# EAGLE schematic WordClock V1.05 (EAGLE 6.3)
PROJECT_LINE1: WordClock; PROJECT_REVISION: 1.05

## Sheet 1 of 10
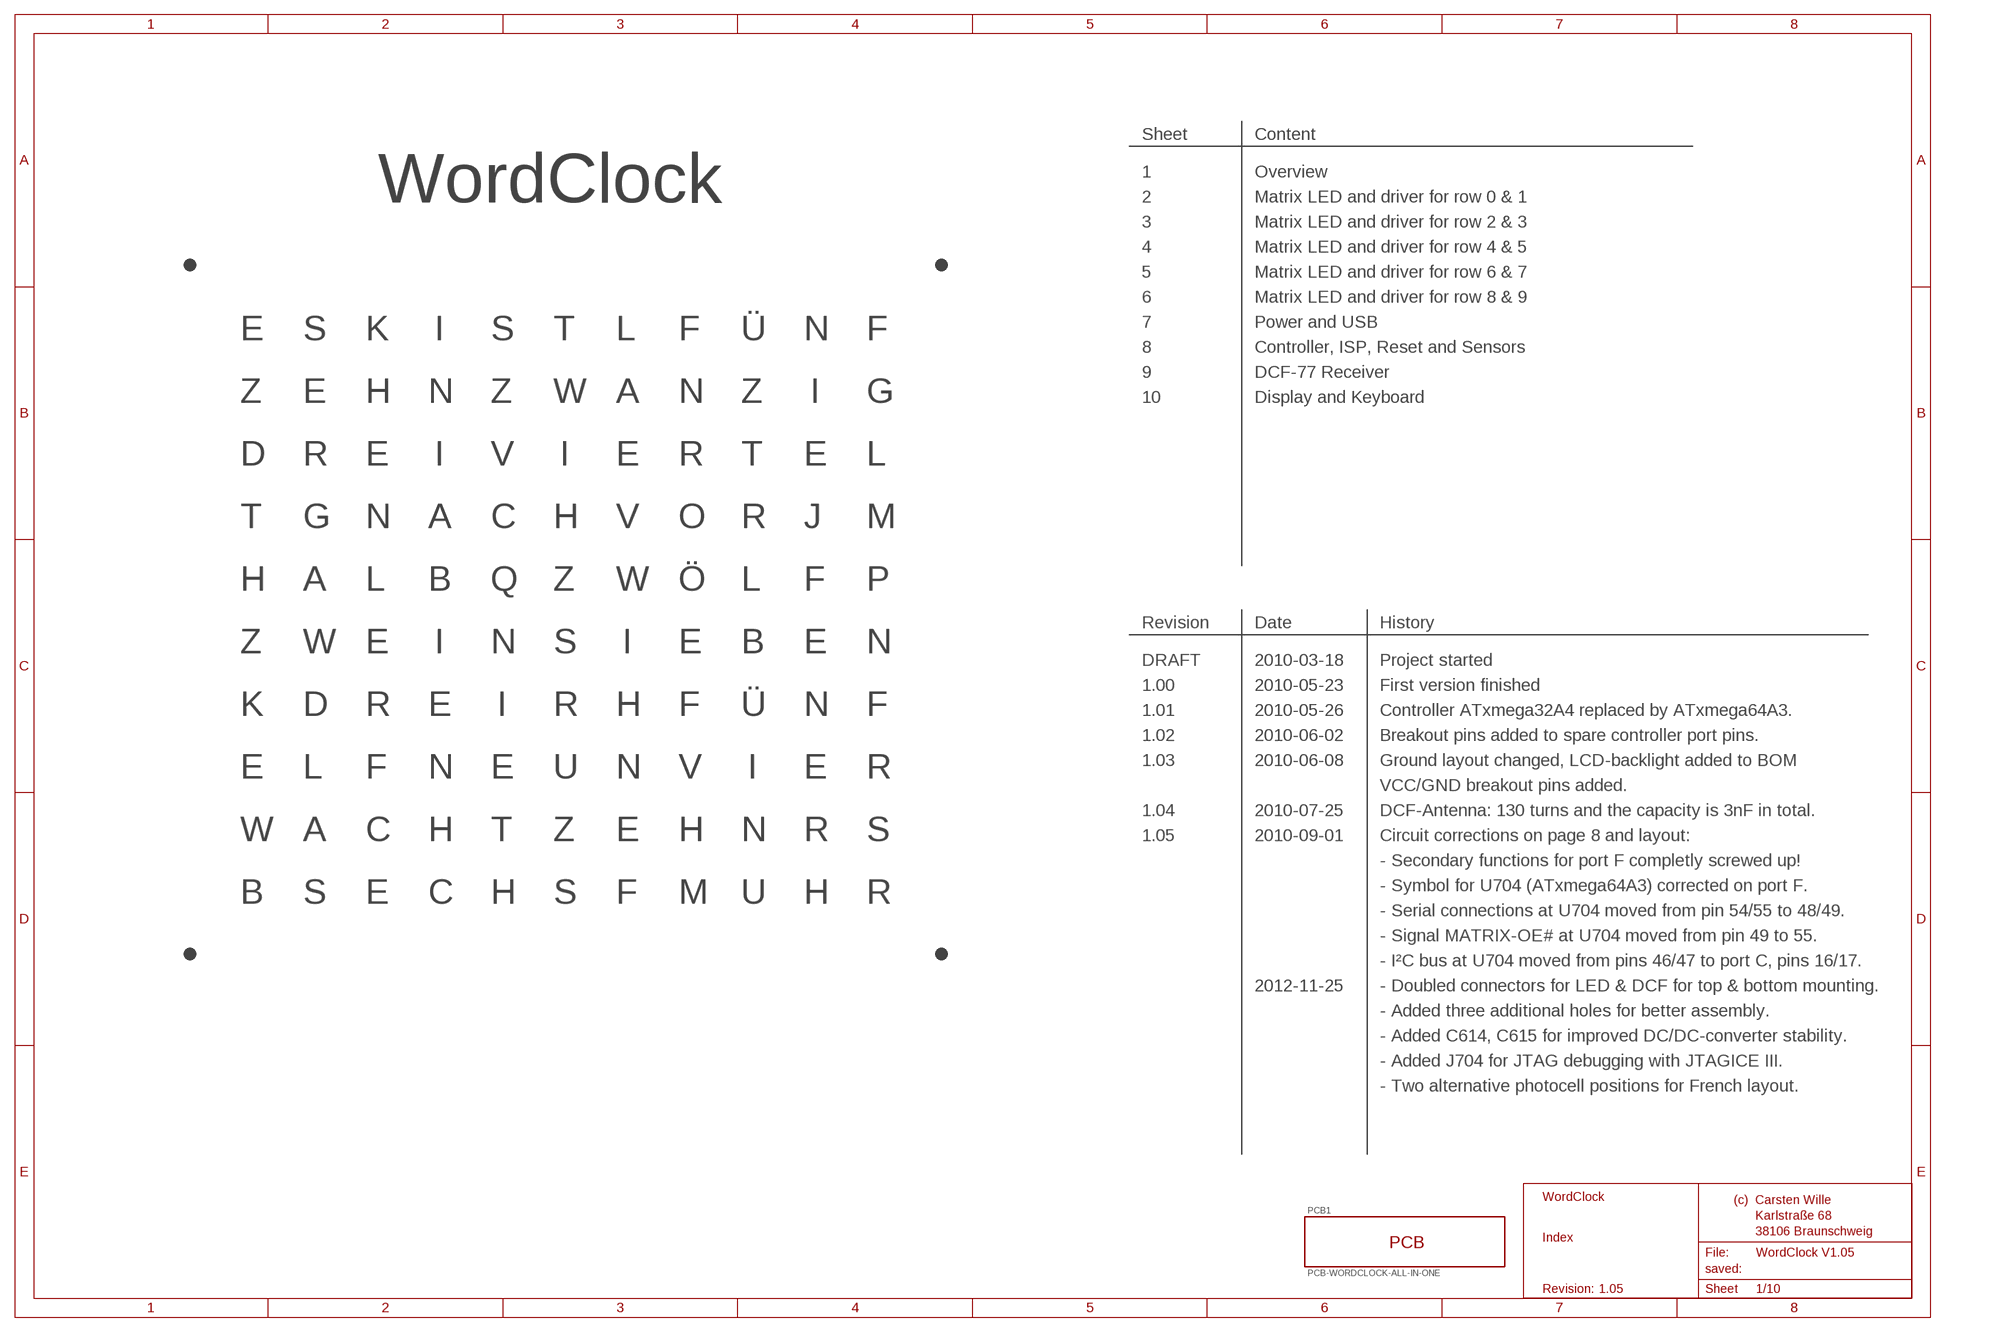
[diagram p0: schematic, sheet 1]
BLATT2 (BLATT-A3-LANDSCAPE_CW): SHEET_LINE1: Index

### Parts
PCB1  PCB-WORDCLOCK-ALL-IN-ONE  PCBWORDCLOCK-ALL-IN-ONE  [WORDCLOCK_S]

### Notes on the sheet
- Sheet | Content
- 1 | Overview
- WordClock | 2 | Matrix LED and driver for row 0 & 1
- 3 | Matrix LED and driver for row 2 & 3
- 4 | Matrix LED and driver for row 4 & 5
- 5 | Matrix LED and driver for row 6 & 7
- 6 | Matrix LED and driver for row 8 & 9
- 7 | Power and USB
- E | S | K | I | S | T | L | F | Ü | N | F
- 8 | Controller, ISP, Reset and Sensors
- 9 | DCF-77 Receiver
- Z | E | H | N | Z | W | A | N | Z | I | G | 10 | Display and Keyboard
- D | R | E | I | V | I | E | R | T | E | L
- T | G | N | A | C | H | V | O | R | J | M
- H | A | L | B | Q | Z | W | Ö | L | F | P
- Revision | Date | History
- Z | W | E | I | N | S | I | E | B | E | N
- DRAFT | 2010-03-18 | Project started
- 1.00 | 2010-05-23 | First version finished
- K | D | R | E | I | R | H | F | Ü | N | F | 1.01 | 2010-05-26 | Controller ATxmega32A4 replaced by ATxmega64A3.
- 1.02 | 2010-06-02 | Breakout pins added to spare controller port pins.
- 1.03 | 2010-06-08 | Ground layout changed, LCD-backlight added to BOM
- E | L | F | N | E | U | N | V | I | E | R
- VCC/GND breakout pins added.
- 1.04 | 2010-07-25 | DCF-Antenna: 130 turns and the capacity is 3nF in total.
- W | A | C | H | T | Z | E | H | N | R | S | 1.05 | 2010-09-01 | Circuit corrections on page 8 and layout:
- - Secondary functions for port F completly screwed up!
- - Symbol for U704 (ATxmega64A3) corrected on port F.
- B | S | E | C | H | S | F | M | U | H | R
- - Serial connections at U704 moved from pin 54/55 to 48/49.
- - Signal MATRIX-OE# at U704 moved from pin 49 to 55.
- - I²C bus at U704 moved from pins 46/47 to port C, pins 16/17.
- 2012-11-25 | - Doubled connectors for LED & DCF for top & bottom mounting.
- - Added three additional holes for better assembly.
- - Added C614, C615 for improved DC/DC-converter stability.
- - Added J704 for JTAG debugging with JTAGICE III.
- - Two alternative photocell positions for French layout.

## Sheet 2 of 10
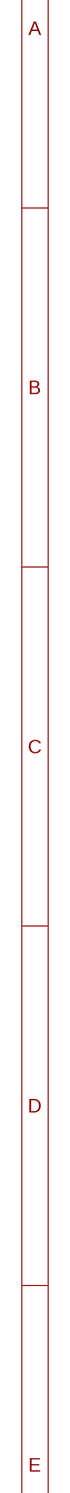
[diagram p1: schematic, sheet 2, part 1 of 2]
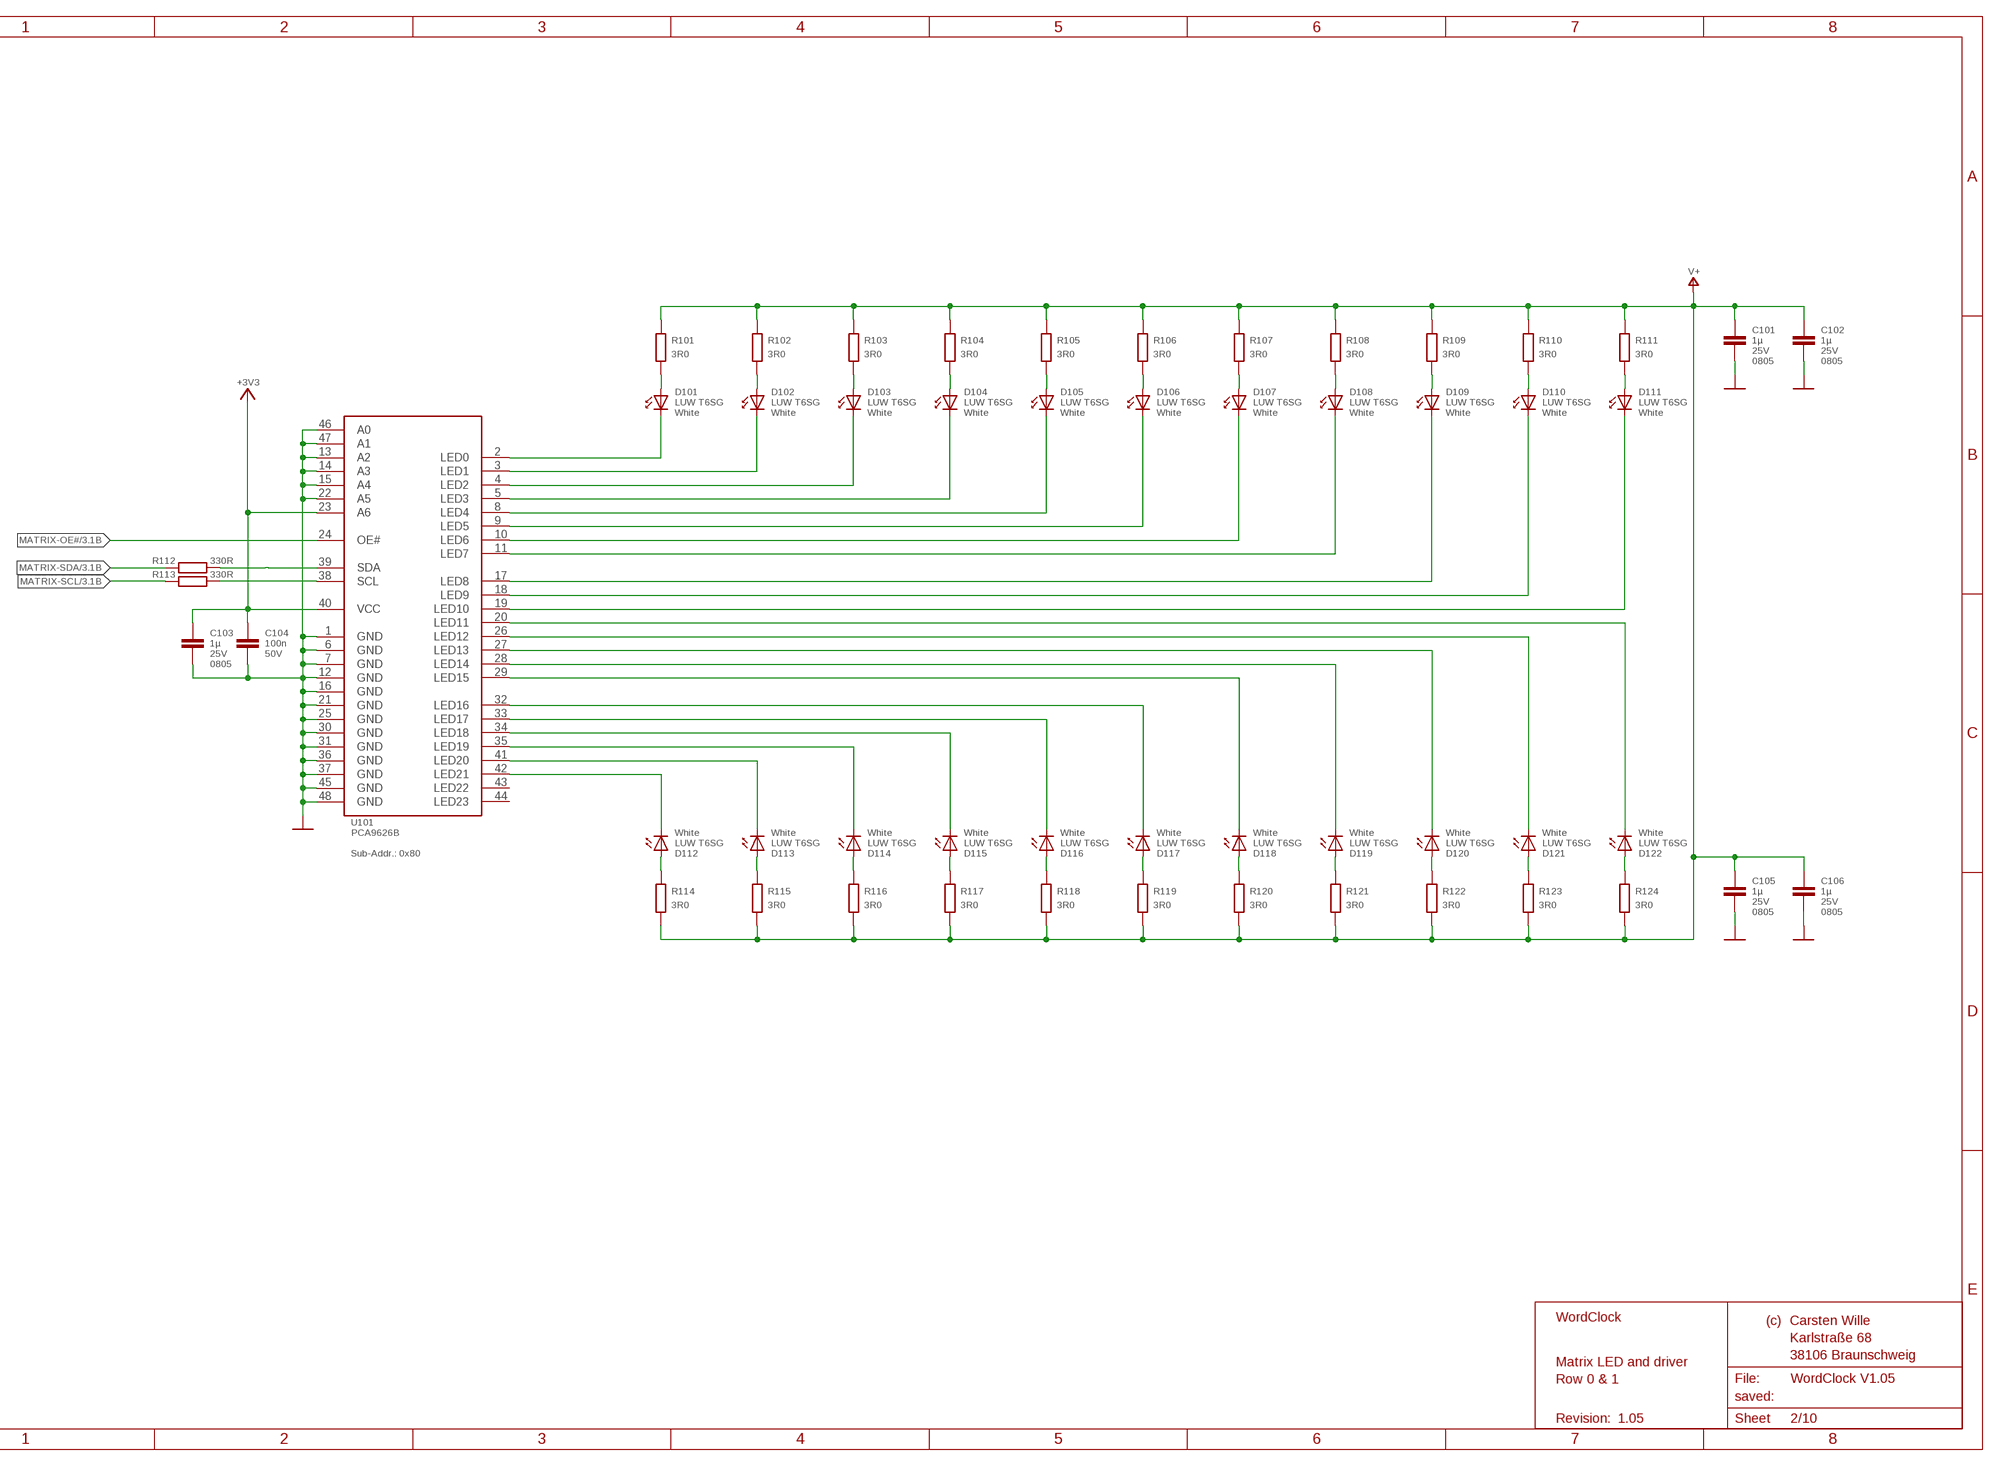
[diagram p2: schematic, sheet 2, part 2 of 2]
BLATT1 (BLATT-A3-LANDSCAPE_CW): SHEET_LINE1: Matrix LED and driver; SHEET_LINE2: Row 0 & 1

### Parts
C101  1E-6-1U-0805  [C0805]
C102  1E-6-1U-0805  [C0805]
C103  1E-6-1U-0805  [C0805]
C104  1E-9-100N-0603  [C0603]
C105  1E-6-1U-0805  [C0805]
C106  1E-6-1U-0805  [C0805]
D101  TOPLED-LUW  [P-LCC-2]
D102  TOPLED-LUW  [P-LCC-2]
D103  TOPLED-LUW  [P-LCC-2]
D104  TOPLED-LUW  [P-LCC-2]
D105  TOPLED-LUW  [P-LCC-2]
D106  TOPLED-LUW  [P-LCC-2]
D107  TOPLED-LUW  [P-LCC-2]
D108  TOPLED-LUW  [P-LCC-2]
D109  TOPLED-LUW  [P-LCC-2]
D110  TOPLED-LUW  [P-LCC-2]
D111  TOPLED-LUW  [P-LCC-2]
D112  TOPLED-LUW  [P-LCC-2]
D113  TOPLED-LUW  [P-LCC-2]
D114  TOPLED-LUW  [P-LCC-2]
D115  TOPLED-LUW  [P-LCC-2]
D116  TOPLED-LUW  [P-LCC-2]
D117  TOPLED-LUW  [P-LCC-2]
D118  TOPLED-LUW  [P-LCC-2]
D119  TOPLED-LUW  [P-LCC-2]
D120  TOPLED-LUW  [P-LCC-2]
D121  TOPLED-LUW  [P-LCC-2]
D122  TOPLED-LUW  [P-LCC-2]
R101  1E0-3,0R-0603  [R0603]
R102  1E0-3,0R-0603  [R0603]
R103  1E0-3,0R-0603  [R0603]
R104  1E0-3,0R-0603  [R0603]
R105  1E0-3,0R-0603  [R0603]
R106  1E0-3,0R-0603  [R0603]
R107  1E0-3,0R-0603  [R0603]
R108  1E0-3,0R-0603  [R0603]
R109  1E0-3,0R-0603  [R0603]
R110  1E0-3,0R-0603  [R0603]
R111  1E0-3,0R-0603  [R0603]
R112  1E2-330R-0603  [R0603]
R113  1E2-330R-0603  [R0603]
R114  1E0-3,0R-0603  [R0603]
R115  1E0-3,0R-0603  [R0603]
R116  1E0-3,0R-0603  [R0603]
R117  1E0-3,0R-0603  [R0603]
R118  1E0-3,0R-0603  [R0603]
R119  1E0-3,0R-0603  [R0603]
R120  1E0-3,0R-0603  [R0603]
R121  1E0-3,0R-0603  [R0603]
R122  1E0-3,0R-0603  [R0603]
R123  1E0-3,0R-0603  [R0603]
R124  1E0-3,0R-0603  [R0603]
U101  PCA9626  [LQFP48]

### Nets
+3V3: C103.1 C104.1 U101.23(A6) U101.40(VCC) ; also sheet 3,4,5,6,7,8
GND: C101.2 C102.2 C103.2 C104.2 C105.2 C106.2 U101.1(GND) U101.6(GND) U101.7(GND) U101.12(GND) U101.13(A2) U101.14(A3) U101.15(A4) U101.16(GND) U101.21(GND) U101.22(A5) U101.25(GND) U101.30(GND) U101.31(GND) U101.36(GND) U101.37(GND) U101.45(GND) U101.46(A0) U101.47(A1) U101.48(GND) ; also sheet 3,4,5,6,7,8
LED0@U1: D101.C U101.2(LED0)
LED1@U1: D102.C U101.3(LED1)
LED2@U1: D103.C U101.4(LED2)
LED3@U1: D104.C U101.5(LED3)
LED4@U1: D105.C U101.8(LED4)
LED5@U1: D106.C U101.9(LED5)
LED6@U1: D107.C U101.10(LED6)
LED7@U1: D108.C U101.11(LED7)
LED8@U1: D109.C U101.17(LED8)
LED9@U1: D110.C U101.18(LED9)
LED10@U1: D111.C U101.19(LED10)
LED11@U1: D122.C U101.20(LED11)
LED12@U1: D121.C U101.26(LED12)
LED13@U1: D120.C U101.27(LED13)
LED14@U1: D119.C U101.28(LED14)
LED15@U1: D118.C U101.29(LED15)
LED16@U1: D117.C U101.32(LED16)
LED17@U1: D116.C U101.33(LED17)
LED18@U1: D115.C U101.34(LED18)
LED19@U1: D114.C U101.35(LED19)
LED20@U1: D113.C U101.41(LED20)
LED21@U1: D112.C U101.42(LED21)
MATRIX-OE#: U101.24(OE#) ; also sheet 3,4,5,6,8
MATRIX-SCL: R113.1 ; also sheet 3,4,5,6,8
MATRIX-SDA: R112.1 ; also sheet 3,4,5,6,8
R1@U1: D101.A R101.2
R2@U1: D102.A R102.2
R3@U1: D103.A R103.2
R4@U1: D104.A R104.2
R5@U1: D105.A R105.2
R6@U1: D106.A R106.2
R7@U1: D107.A R107.2
R8@U1: D108.A R108.2
R9@U1: D109.A R109.2
R10@U1: D110.A R110.2
R11@U1: D111.A R111.2
R12@U1: D112.A R114.1
R13@U1: D113.A R115.1
R14@U1: D114.A R116.1
R15@U1: D115.A R117.1
R16@U1: D116.A R118.1
R17@U1: D117.A R119.1
R18@U1: D118.A R120.1
R19@U1: D119.A R121.1
R20@U1: D120.A R122.1
R21@U1: D121.A R123.1
R22@U1: D122.A R124.1
SCL@U1: R113.2 U101.38(SCL)
SDA@U1: R112.2 U101.39(SDA)
V+: C101.1 C102.1 C105.1 C106.1 R101.1 R102.1 R103.1 R104.1 R105.1 R106.1 R107.1 R108.1 R109.1 R110.1 R111.1 R114.2 R115.2 R116.2 R117.2 R118.2 R119.2 R120.2 R121.2 R122.2 R123.2 R124.2 ; also sheet 3,4,5,6,7
Unconnected: U101.43(LED22) U101.44(LED23)

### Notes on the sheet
- Sub-Addr.: 0x80

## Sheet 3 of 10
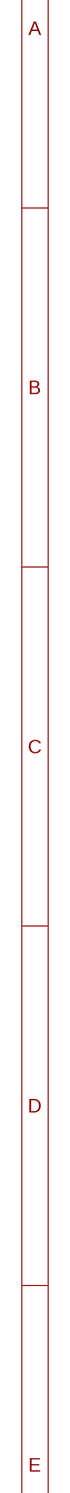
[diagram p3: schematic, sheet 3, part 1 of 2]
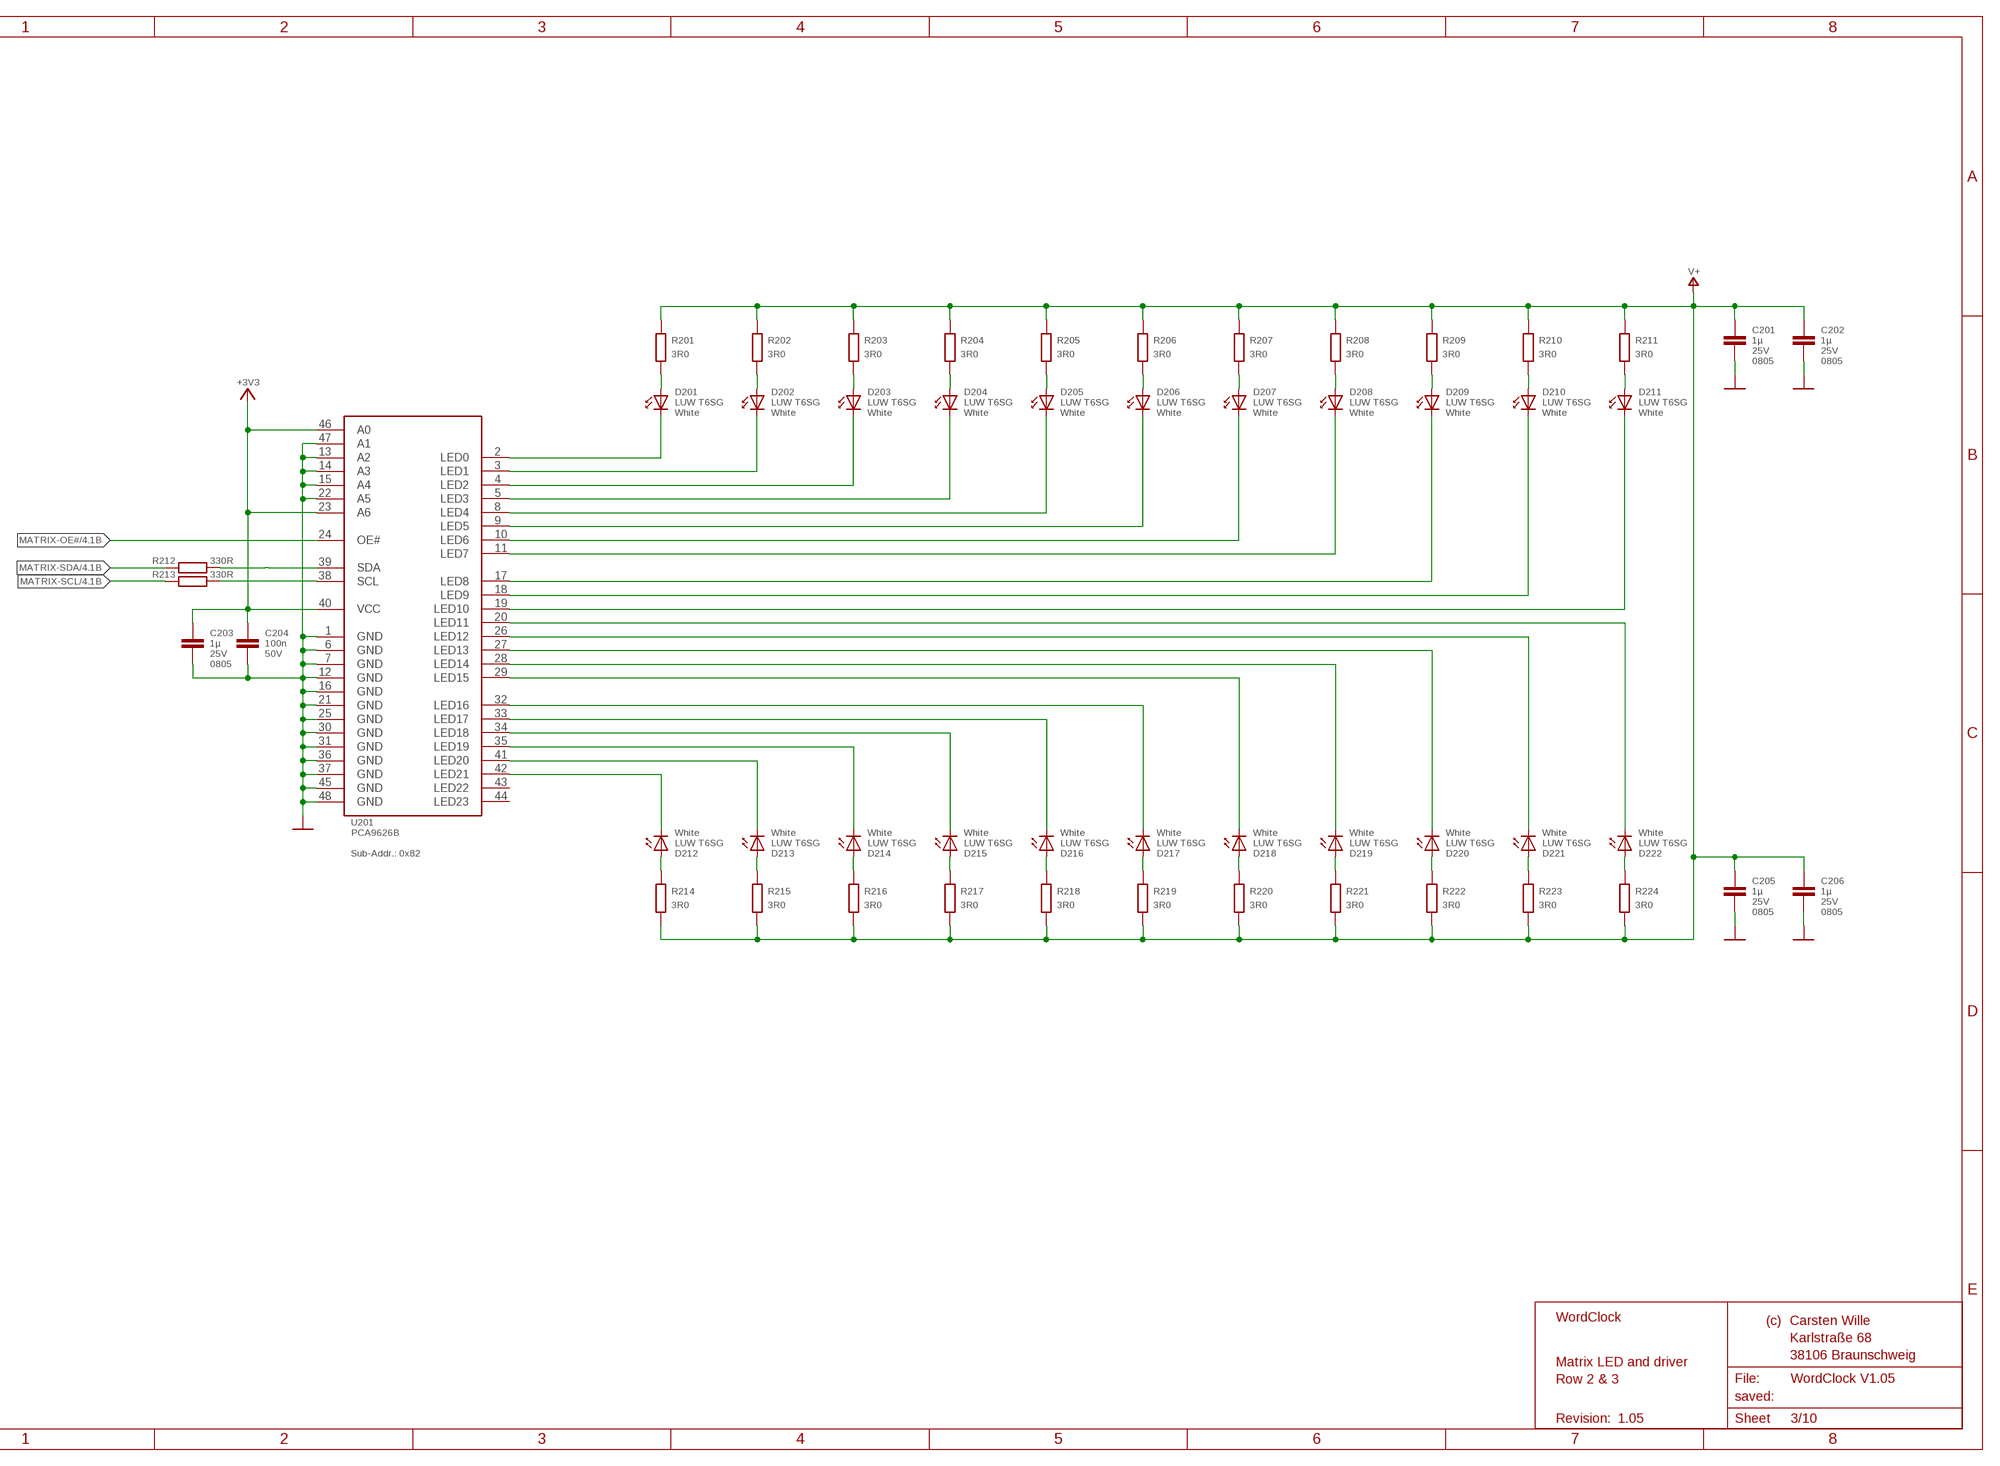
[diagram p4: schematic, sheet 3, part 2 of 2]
BLATT3 (BLATT-A3-LANDSCAPE_CW): SHEET_LINE1: Matrix LED and driver; SHEET_LINE2: Row 2 & 3

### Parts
C201  1E-6-1U-0805  [C0805]
C202  1E-6-1U-0805  [C0805]
C203  1E-6-1U-0805  [C0805]
C204  1E-9-100N-0603  [C0603]
C205  1E-6-1U-0805  [C0805]
C206  1E-6-1U-0805  [C0805]
D201  TOPLED-LUW  [P-LCC-2]
D202  TOPLED-LUW  [P-LCC-2]
D203  TOPLED-LUW  [P-LCC-2]
D204  TOPLED-LUW  [P-LCC-2]
D205  TOPLED-LUW  [P-LCC-2]
D206  TOPLED-LUW  [P-LCC-2]
D207  TOPLED-LUW  [P-LCC-2]
D208  TOPLED-LUW  [P-LCC-2]
D209  TOPLED-LUW  [P-LCC-2]
D210  TOPLED-LUW  [P-LCC-2]
D211  TOPLED-LUW  [P-LCC-2]
D212  TOPLED-LUW  [P-LCC-2]
D213  TOPLED-LUW  [P-LCC-2]
D214  TOPLED-LUW  [P-LCC-2]
D215  TOPLED-LUW  [P-LCC-2]
D216  TOPLED-LUW  [P-LCC-2]
D217  TOPLED-LUW  [P-LCC-2]
D218  TOPLED-LUW  [P-LCC-2]
D219  TOPLED-LUW  [P-LCC-2]
D220  TOPLED-LUW  [P-LCC-2]
D221  TOPLED-LUW  [P-LCC-2]
D222  TOPLED-LUW  [P-LCC-2]
R201  1E0-3,0R-0603  [R0603]
R202  1E0-3,0R-0603  [R0603]
R203  1E0-3,0R-0603  [R0603]
R204  1E0-3,0R-0603  [R0603]
R205  1E0-3,0R-0603  [R0603]
R206  1E0-3,0R-0603  [R0603]
R207  1E0-3,0R-0603  [R0603]
R208  1E0-3,0R-0603  [R0603]
R209  1E0-3,0R-0603  [R0603]
R210  1E0-3,0R-0603  [R0603]
R211  1E0-3,0R-0603  [R0603]
R212  1E2-330R-0603  [R0603]
R213  1E2-330R-0603  [R0603]
R214  1E0-3,0R-0603  [R0603]
R215  1E0-3,0R-0603  [R0603]
R216  1E0-3,0R-0603  [R0603]
R217  1E0-3,0R-0603  [R0603]
R218  1E0-3,0R-0603  [R0603]
R219  1E0-3,0R-0603  [R0603]
R220  1E0-3,0R-0603  [R0603]
R221  1E0-3,0R-0603  [R0603]
R222  1E0-3,0R-0603  [R0603]
R223  1E0-3,0R-0603  [R0603]
R224  1E0-3,0R-0603  [R0603]
U201  PCA9626  [LQFP48]

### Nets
+3V3: C203.1 C204.1 U201.23(A6) U201.40(VCC) U201.46(A0) ; also sheet 2,4,5,6,7,8
GND: C201.2 C202.2 C203.2 C204.2 C205.2 C206.2 U201.1(GND) U201.6(GND) U201.7(GND) U201.12(GND) U201.13(A2) U201.14(A3) U201.15(A4) U201.16(GND) U201.21(GND) U201.22(A5) U201.25(GND) U201.30(GND) U201.31(GND) U201.36(GND) U201.37(GND) U201.45(GND) U201.47(A1) U201.48(GND) ; also sheet 2,4,5,6,7,8
LED0@U2: D201.C U201.2(LED0)
LED1@U2: D202.C U201.3(LED1)
LED2@U2: D203.C U201.4(LED2)
LED3@U2: D204.C U201.5(LED3)
LED4@U2: D205.C U201.8(LED4)
LED5@U2: D206.C U201.9(LED5)
LED6@U2: D207.C U201.10(LED6)
LED7@U2: D208.C U201.11(LED7)
LED8@U2: D209.C U201.17(LED8)
LED9@U2: D210.C U201.18(LED9)
LED10@U2: D211.C U201.19(LED10)
LED11@U2: D222.C U201.20(LED11)
LED12@U2: D221.C U201.26(LED12)
LED13@U2: D220.C U201.27(LED13)
LED14@U2: D219.C U201.28(LED14)
LED15@U2: D218.C U201.29(LED15)
LED16@U2: D217.C U201.32(LED16)
LED17@U2: D216.C U201.33(LED17)
LED18@U2: D215.C U201.34(LED18)
LED19@U2: D214.C U201.35(LED19)
LED20@U2: D213.C U201.41(LED20)
LED21@U2: D212.C U201.42(LED21)
MATRIX-OE#: U201.24(OE#) ; also sheet 2,4,5,6,8
MATRIX-SCL: R213.1 ; also sheet 2,4,5,6,8
MATRIX-SDA: R212.1 ; also sheet 2,4,5,6,8
R1@U2: D201.A R201.2
R2@U2: D202.A R202.2
R3@U2: D203.A R203.2
R4@U2: D204.A R204.2
R5@U2: D205.A R205.2
R6@U2: D206.A R206.2
R7@U2: D207.A R207.2
R8@U2: D208.A R208.2
R9@U2: D209.A R209.2
R10@U2: D210.A R210.2
R11@U2: D211.A R211.2
R12@U2: D212.A R214.1
R13@U2: D213.A R215.1
R14@U2: D214.A R216.1
R15@U2: D215.A R217.1
R16@U2: D216.A R218.1
R17@U2: D217.A R219.1
R18@U2: D218.A R220.1
R19@U2: D219.A R221.1
R20@U2: D220.A R222.1
R21@U2: D221.A R223.1
R22@U2: D222.A R224.1
SCL@U2: R213.2 U201.38(SCL)
SDA@U2: R212.2 U201.39(SDA)
V+: C201.1 C202.1 C205.1 C206.1 R201.1 R202.1 R203.1 R204.1 R205.1 R206.1 R207.1 R208.1 R209.1 R210.1 R211.1 R214.2 R215.2 R216.2 R217.2 R218.2 R219.2 R220.2 R221.2 R222.2 R223.2 R224.2 ; also sheet 2,4,5,6,7
Unconnected: U201.43(LED22) U201.44(LED23)

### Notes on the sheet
- Sub-Addr.: 0x82

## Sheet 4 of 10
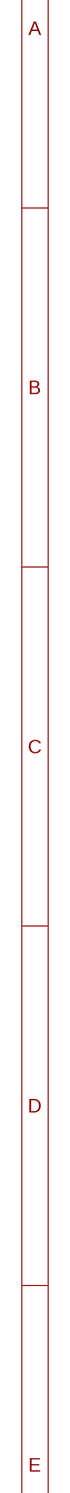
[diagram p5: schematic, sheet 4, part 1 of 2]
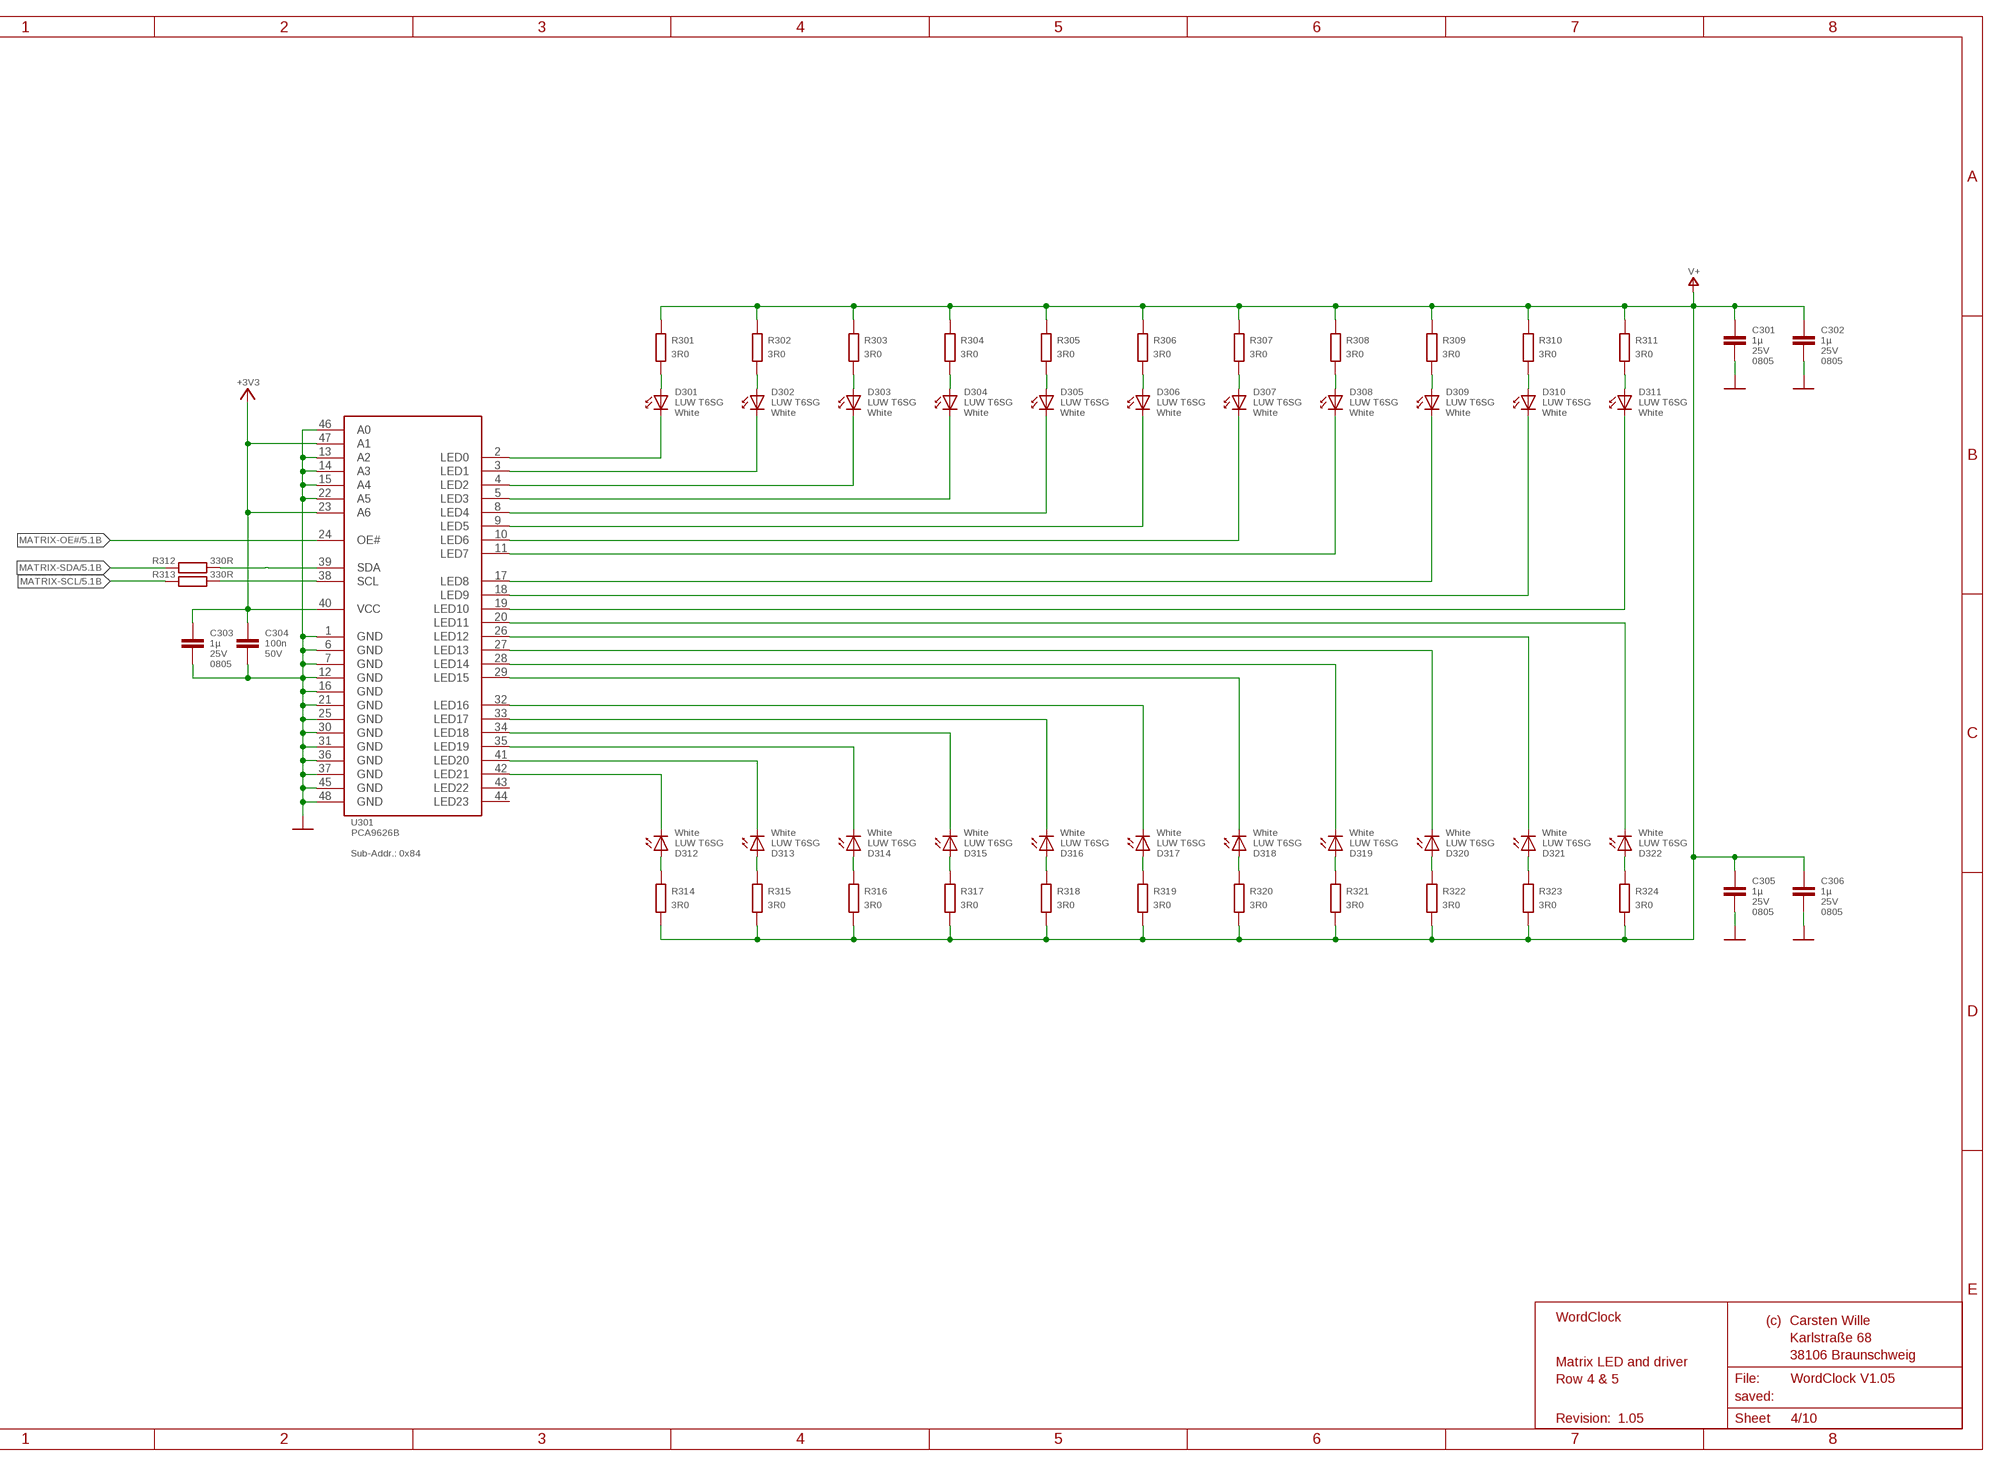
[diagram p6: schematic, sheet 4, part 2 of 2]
BLATT4 (BLATT-A3-LANDSCAPE_CW): SHEET_LINE1: Matrix LED and driver; SHEET_LINE2: Row 4 & 5

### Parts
C301  1E-6-1U-0805  [C0805]
C302  1E-6-1U-0805  [C0805]
C303  1E-6-1U-0805  [C0805]
C304  1E-9-100N-0603  [C0603]
C305  1E-6-1U-0805  [C0805]
C306  1E-6-1U-0805  [C0805]
D301  TOPLED-LUW  [P-LCC-2]
D302  TOPLED-LUW  [P-LCC-2]
D303  TOPLED-LUW  [P-LCC-2]
D304  TOPLED-LUW  [P-LCC-2]
D305  TOPLED-LUW  [P-LCC-2]
D306  TOPLED-LUW  [P-LCC-2]
D307  TOPLED-LUW  [P-LCC-2]
D308  TOPLED-LUW  [P-LCC-2]
D309  TOPLED-LUW  [P-LCC-2]
D310  TOPLED-LUW  [P-LCC-2]
D311  TOPLED-LUW  [P-LCC-2]
D312  TOPLED-LUW  [P-LCC-2]
D313  TOPLED-LUW  [P-LCC-2]
D314  TOPLED-LUW  [P-LCC-2]
D315  TOPLED-LUW  [P-LCC-2]
D316  TOPLED-LUW  [P-LCC-2]
D317  TOPLED-LUW  [P-LCC-2]
D318  TOPLED-LUW  [P-LCC-2]
D319  TOPLED-LUW  [P-LCC-2]
D320  TOPLED-LUW  [P-LCC-2]
D321  TOPLED-LUW  [P-LCC-2]
D322  TOPLED-LUW  [P-LCC-2]
R301  1E0-3,0R-0603  [R0603]
R302  1E0-3,0R-0603  [R0603]
R303  1E0-3,0R-0603  [R0603]
R304  1E0-3,0R-0603  [R0603]
R305  1E0-3,0R-0603  [R0603]
R306  1E0-3,0R-0603  [R0603]
R307  1E0-3,0R-0603  [R0603]
R308  1E0-3,0R-0603  [R0603]
R309  1E0-3,0R-0603  [R0603]
R310  1E0-3,0R-0603  [R0603]
R311  1E0-3,0R-0603  [R0603]
R312  1E2-330R-0603  [R0603]
R313  1E2-330R-0603  [R0603]
R314  1E0-3,0R-0603  [R0603]
R315  1E0-3,0R-0603  [R0603]
R316  1E0-3,0R-0603  [R0603]
R317  1E0-3,0R-0603  [R0603]
R318  1E0-3,0R-0603  [R0603]
R319  1E0-3,0R-0603  [R0603]
R320  1E0-3,0R-0603  [R0603]
R321  1E0-3,0R-0603  [R0603]
R322  1E0-3,0R-0603  [R0603]
R323  1E0-3,0R-0603  [R0603]
R324  1E0-3,0R-0603  [R0603]
U301  PCA9626  [LQFP48]

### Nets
+3V3: C303.1 C304.1 U301.23(A6) U301.40(VCC) U301.47(A1) ; also sheet 2,3,5,6,7,8
GND: C301.2 C302.2 C303.2 C304.2 C305.2 C306.2 U301.1(GND) U301.6(GND) U301.7(GND) U301.12(GND) U301.13(A2) U301.14(A3) U301.15(A4) U301.16(GND) U301.21(GND) U301.22(A5) U301.25(GND) U301.30(GND) U301.31(GND) U301.36(GND) U301.37(GND) U301.45(GND) U301.46(A0) U301.48(GND) ; also sheet 2,3,5,6,7,8
LED0@U3: D301.C U301.2(LED0)
LED1@U3: D302.C U301.3(LED1)
LED2@U3: D303.C U301.4(LED2)
LED3@U3: D304.C U301.5(LED3)
LED4@U3: D305.C U301.8(LED4)
LED5@U3: D306.C U301.9(LED5)
LED6@U3: D307.C U301.10(LED6)
LED7@U3: D308.C U301.11(LED7)
LED8@U3: D309.C U301.17(LED8)
LED9@U3: D310.C U301.18(LED9)
LED10@U3: D311.C U301.19(LED10)
LED11@U3: D322.C U301.20(LED11)
LED12@U3: D321.C U301.26(LED12)
LED13@U3: D320.C U301.27(LED13)
LED14@U3: D319.C U301.28(LED14)
LED15@U3: D318.C U301.29(LED15)
LED16@U3: D317.C U301.32(LED16)
LED17@U3: D316.C U301.33(LED17)
LED18@U3: D315.C U301.34(LED18)
LED19@U3: D314.C U301.35(LED19)
LED20@U3: D313.C U301.41(LED20)
LED21@U3: D312.C U301.42(LED21)
MATRIX-OE#: U301.24(OE#) ; also sheet 2,3,5,6,8
MATRIX-SCL: R313.1 ; also sheet 2,3,5,6,8
MATRIX-SDA: R312.1 ; also sheet 2,3,5,6,8
R1@U3: D301.A R301.2
R2@U3: D302.A R302.2
R3@U3: D303.A R303.2
R4@U3: D304.A R304.2
R5@U3: D305.A R305.2
R6@U3: D306.A R306.2
R7@U3: D307.A R307.2
R8@U3: D308.A R308.2
R9@U3: D309.A R309.2
R10@U3: D310.A R310.2
R11@U3: D311.A R311.2
R12@U3: D312.A R314.1
R13@U3: D313.A R315.1
R14@U3: D314.A R316.1
R15@U3: D315.A R317.1
R16@U3: D316.A R318.1
R17@U3: D317.A R319.1
R18@U3: D318.A R320.1
R19@U3: D319.A R321.1
R20@U3: D320.A R322.1
R21@U3: D321.A R323.1
R22@U3: D322.A R324.1
SCL@U3: R313.2 U301.38(SCL)
SDA@U3: R312.2 U301.39(SDA)
V+: C301.1 C302.1 C305.1 C306.1 R301.1 R302.1 R303.1 R304.1 R305.1 R306.1 R307.1 R308.1 R309.1 R310.1 R311.1 R314.2 R315.2 R316.2 R317.2 R318.2 R319.2 R320.2 R321.2 R322.2 R323.2 R324.2 ; also sheet 2,3,5,6,7
Unconnected: U301.43(LED22) U301.44(LED23)

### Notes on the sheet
- Sub-Addr.: 0x84

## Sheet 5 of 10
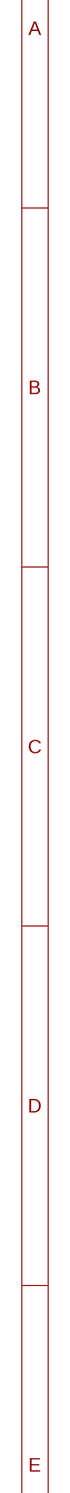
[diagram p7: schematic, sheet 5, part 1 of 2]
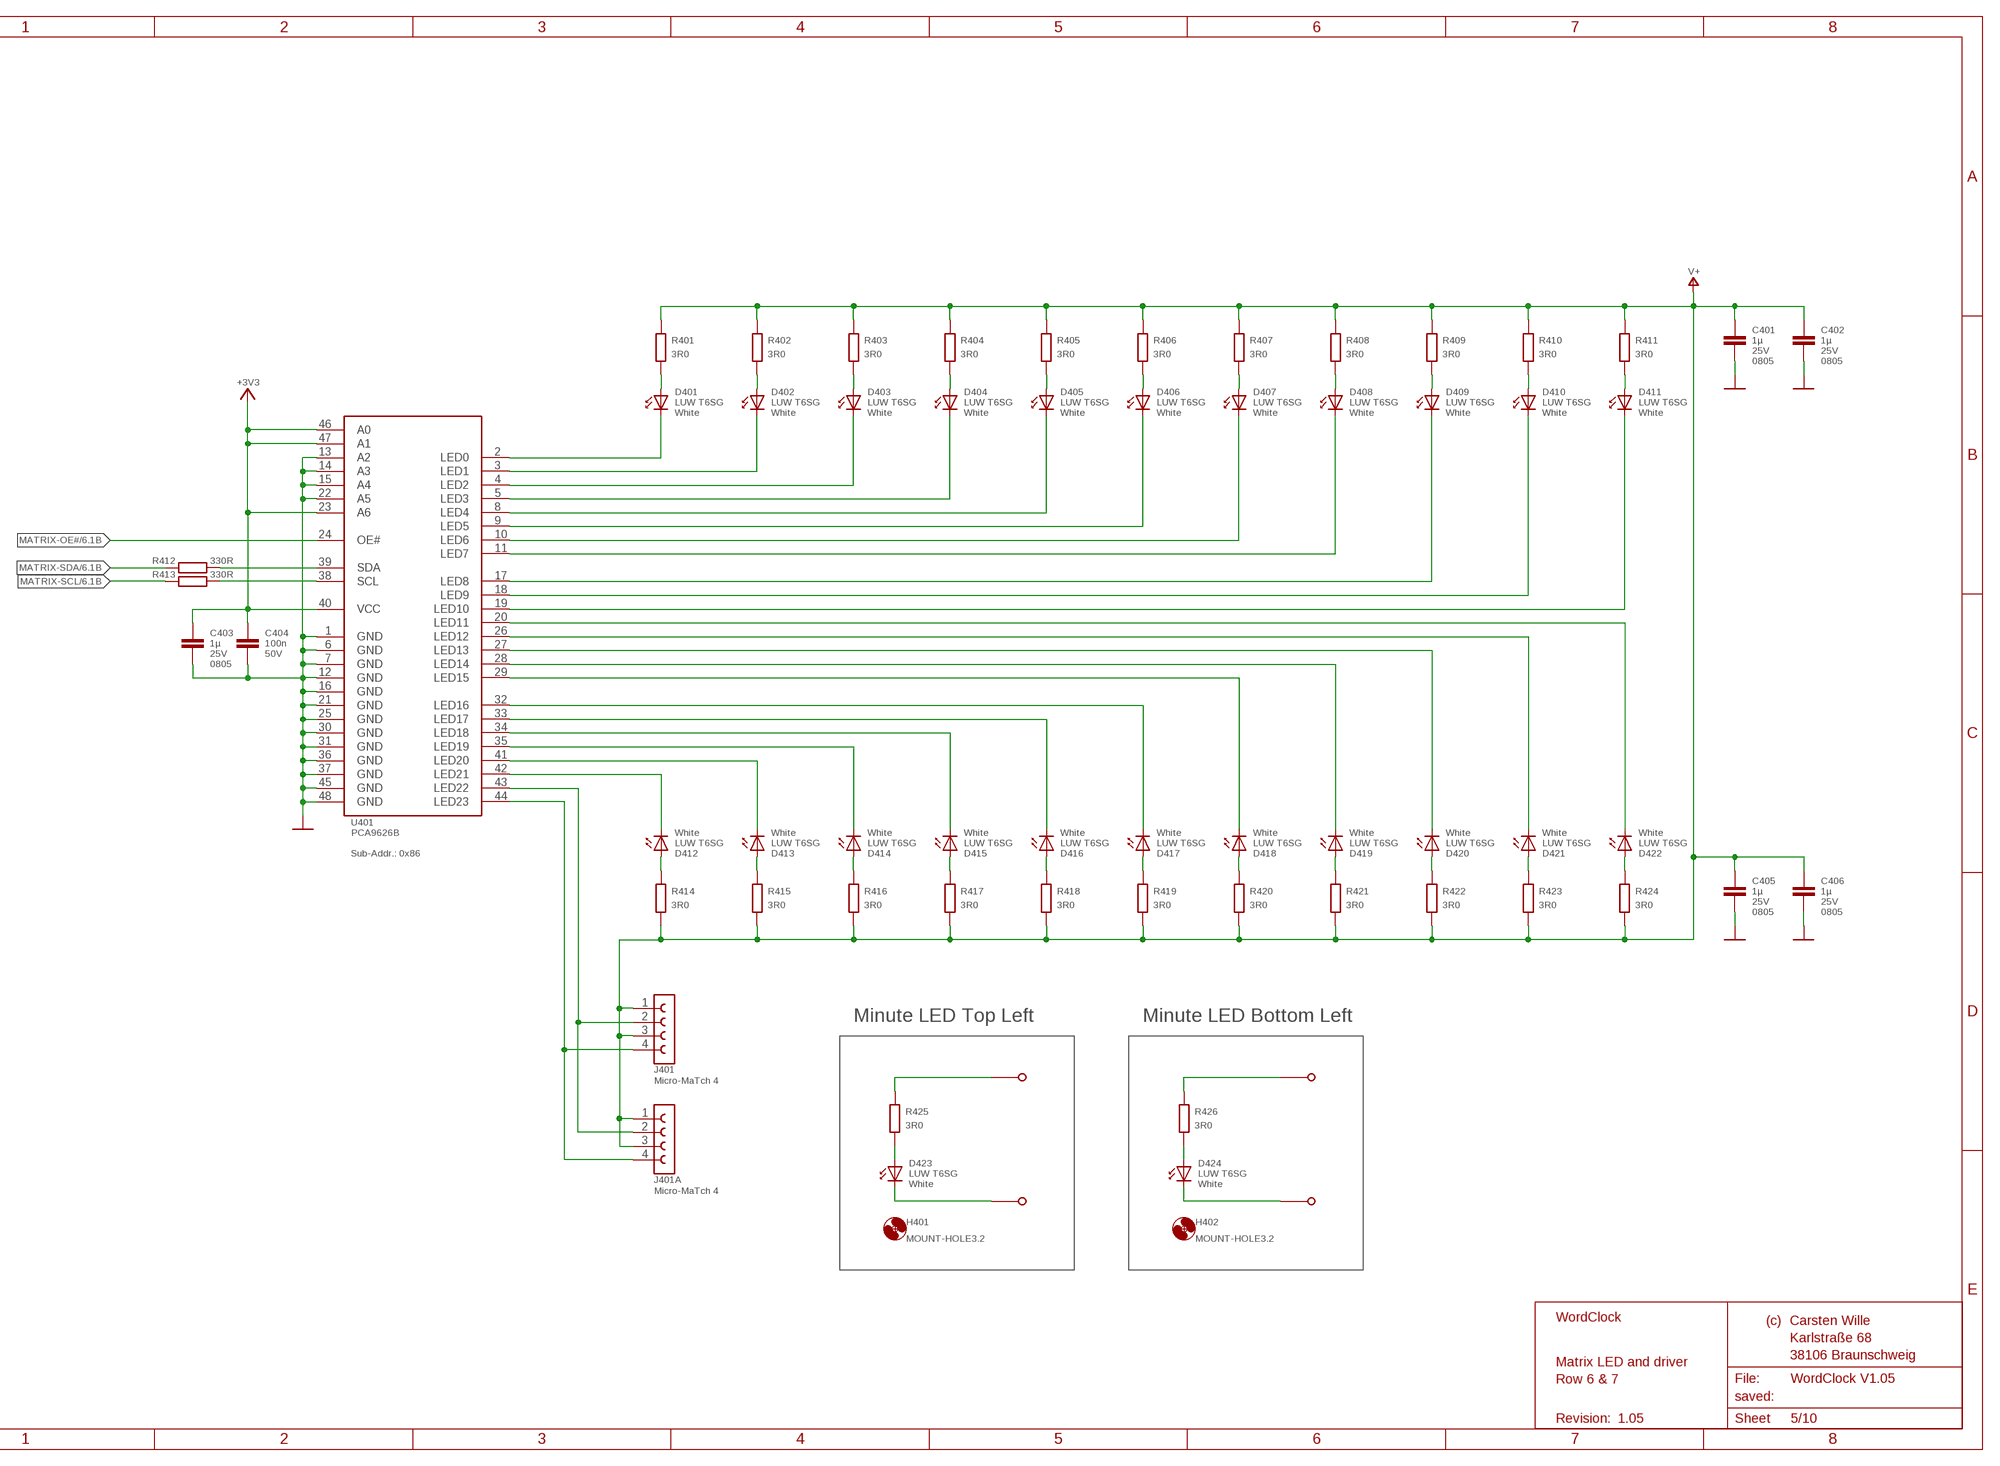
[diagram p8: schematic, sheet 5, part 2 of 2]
BLATT5 (BLATT-A3-LANDSCAPE_CW): SHEET_LINE1: Matrix LED and driver; SHEET_LINE2: Row 6 & 7

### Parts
C401  1E-6-1U-0805  [C0805]
C402  1E-6-1U-0805  [C0805]
C403  1E-6-1U-0805  [C0805]
C404  1E-9-100N-0603  [C0603]
C405  1E-6-1U-0805  [C0805]
C406  1E-6-1U-0805  [C0805]
D401  TOPLED-LUW  [P-LCC-2]
D402  TOPLED-LUW  [P-LCC-2]
D403  TOPLED-LUW  [P-LCC-2]
D404  TOPLED-LUW  [P-LCC-2]
D405  TOPLED-LUW  [P-LCC-2]
D406  TOPLED-LUW  [P-LCC-2]
D407  TOPLED-LUW  [P-LCC-2]
D408  TOPLED-LUW  [P-LCC-2]
D409  TOPLED-LUW  [P-LCC-2]
D410  TOPLED-LUW  [P-LCC-2]
D411  TOPLED-LUW  [P-LCC-2]
D412  TOPLED-LUW  [P-LCC-2]
D413  TOPLED-LUW  [P-LCC-2]
D414  TOPLED-LUW  [P-LCC-2]
D415  TOPLED-LUW  [P-LCC-2]
D416  TOPLED-LUW  [P-LCC-2]
D417  TOPLED-LUW  [P-LCC-2]
D418  TOPLED-LUW  [P-LCC-2]
D419  TOPLED-LUW  [P-LCC-2]
D420  TOPLED-LUW  [P-LCC-2]
D421  TOPLED-LUW  [P-LCC-2]
D422  TOPLED-LUW  [P-LCC-2]
D423  TOPLED-LUW  [P-LCC-2]
D424  TOPLED-LUW  [P-LCC-2]
H401  MOUNT-HOLE3.2  [3,2]
H402  MOUNT-HOLE3.2  [3,2]
J401  MICRO-MATCH-4  [MICRO-MATCH-4]
J401A  MICRO-MATCH-4  [MICRO-MATCH-4]
R401  1E0-3,0R-0603  [R0603]
R402  1E0-3,0R-0603  [R0603]
R403  1E0-3,0R-0603  [R0603]
R404  1E0-3,0R-0603  [R0603]
R405  1E0-3,0R-0603  [R0603]
R406  1E0-3,0R-0603  [R0603]
R407  1E0-3,0R-0603  [R0603]
R408  1E0-3,0R-0603  [R0603]
R409  1E0-3,0R-0603  [R0603]
R410  1E0-3,0R-0603  [R0603]
R411  1E0-3,0R-0603  [R0603]
R412  1E2-330R-0603  [R0603]
R413  1E2-330R-0603  [R0603]
R414  1E0-3,0R-0603  [R0603]
R415  1E0-3,0R-0603  [R0603]
R416  1E0-3,0R-0603  [R0603]
R417  1E0-3,0R-0603  [R0603]
R418  1E0-3,0R-0603  [R0603]
R419  1E0-3,0R-0603  [R0603]
R420  1E0-3,0R-0603  [R0603]
R421  1E0-3,0R-0603  [R0603]
R422  1E0-3,0R-0603  [R0603]
R423  1E0-3,0R-0603  [R0603]
R424  1E0-3,0R-0603  [R0603]
R425  1E0-3,0R-0603  [R0603]
R426  1E0-3,0R-0603  [R0603]
U401  PCA9626  [LQFP48]
X401  SINGLE-PIN-40MIL  [SINGLE-PIN_BIG]
X402  SINGLE-PIN-40MIL  [SINGLE-PIN_BIG]
X403  SINGLE-PIN-40MIL  [SINGLE-PIN_BIG]
X404  SINGLE-PIN-40MIL  [SINGLE-PIN_BIG]

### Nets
+3V3: C403.1 C404.1 U401.23(A6) U401.40(VCC) U401.46(A0) U401.47(A1) ; also sheet 2,3,4,6,7,8
GND: C401.2 C402.2 C403.2 C404.2 C405.2 C406.2 U401.1(GND) U401.6(GND) U401.7(GND) U401.12(GND) U401.13(A2) U401.14(A3) U401.15(A4) U401.16(GND) U401.21(GND) U401.22(A5) U401.25(GND) U401.30(GND) U401.31(GND) U401.36(GND) U401.37(GND) U401.45(GND) U401.48(GND) ; also sheet 2,3,4,6,7,8
LED0@U4: D401.C U401.2(LED0)
LED1@U4: D402.C U401.3(LED1)
LED2@U4: D403.C U401.4(LED2)
LED3@U4: D404.C U401.5(LED3)
LED4@U4: D405.C U401.8(LED4)
LED5@U4: D406.C U401.9(LED5)
LED6@U4: D407.C U401.10(LED6)
LED7@U4: D408.C U401.11(LED7)
LED8@U4: D409.C U401.17(LED8)
LED9@U4: D410.C U401.18(LED9)
LED10@U4: D411.C U401.19(LED10)
LED11@U4: D422.C U401.20(LED11)
LED12@U4: D421.C U401.26(LED12)
LED13@U4: D420.C U401.27(LED13)
LED14@U4: D419.C U401.28(LED14)
LED15@U4: D418.C U401.29(LED15)
LED16@U4: D417.C U401.32(LED16)
LED17@U4: D416.C U401.33(LED17)
LED18@U4: D415.C U401.34(LED18)
LED19@U4: D414.C U401.35(LED19)
LED20@U4: D413.C U401.41(LED20)
LED21@U4: D412.C U401.42(LED21)
MATRIX-OE#: U401.24(OE#) ; also sheet 2,3,4,6,8
MATRIX-SCL: R413.1 ; also sheet 2,3,4,6,8
MATRIX-SDA: R412.1 ; also sheet 2,3,4,6,8
N$48: J401.2 J401A.2 U401.43(LED22)
N$54: J401.4 J401A.4 U401.44(LED23)
N$55: D423.C X403.1
N$56: D423.A R425.2
N$57: R425.1 X401.1
N$58: R426.1 X402.1
N$60: D424.C X404.1
N$62: D424.A R426.2
R1@U4: D401.A R401.2
R2@U4: D402.A R402.2
R3@U4: D403.A R403.2
R4@U4: D404.A R404.2
R5@U4: D405.A R405.2
R6@U4: D406.A R406.2
R7@U4: D407.A R407.2
R8@U4: D408.A R408.2
R9@U4: D409.A R409.2
R10@U4: D410.A R410.2
R11@U4: D411.A R411.2
R12@U4: D412.A R414.1
R13@U4: D413.A R415.1
R14@U4: D414.A R416.1
R15@U4: D415.A R417.1
R16@U4: D416.A R418.1
R17@U4: D417.A R419.1
R18@U4: D418.A R420.1
R19@U4: D419.A R421.1
R20@U4: D420.A R422.1
R21@U4: D421.A R423.1
R22@U4: D422.A R424.1
SCL@U4: R413.2 U401.38(SCL)
SDA@U4: R412.2 U401.39(SDA)
V+: C401.1 C402.1 C405.1 C406.1 J401.1 J401.3 J401A.1 J401A.3 R401.1 R402.1 R403.1 R404.1 R405.1 R406.1 R407.1 R408.1 R409.1 R410.1 R411.1 R414.2 R415.2 R416.2 R417.2 R418.2 R419.2 R420.2 R421.2 R422.2 R423.2 R424.2 ; also sheet 2,3,4,6,7

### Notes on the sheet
- Sub-Addr.: 0x86
- Minute LED Top Left | Minute LED Bottom Left

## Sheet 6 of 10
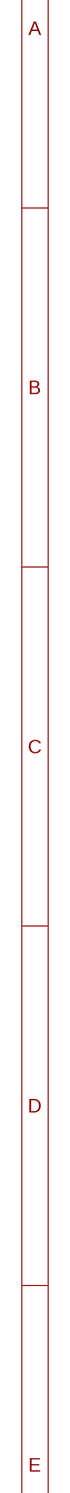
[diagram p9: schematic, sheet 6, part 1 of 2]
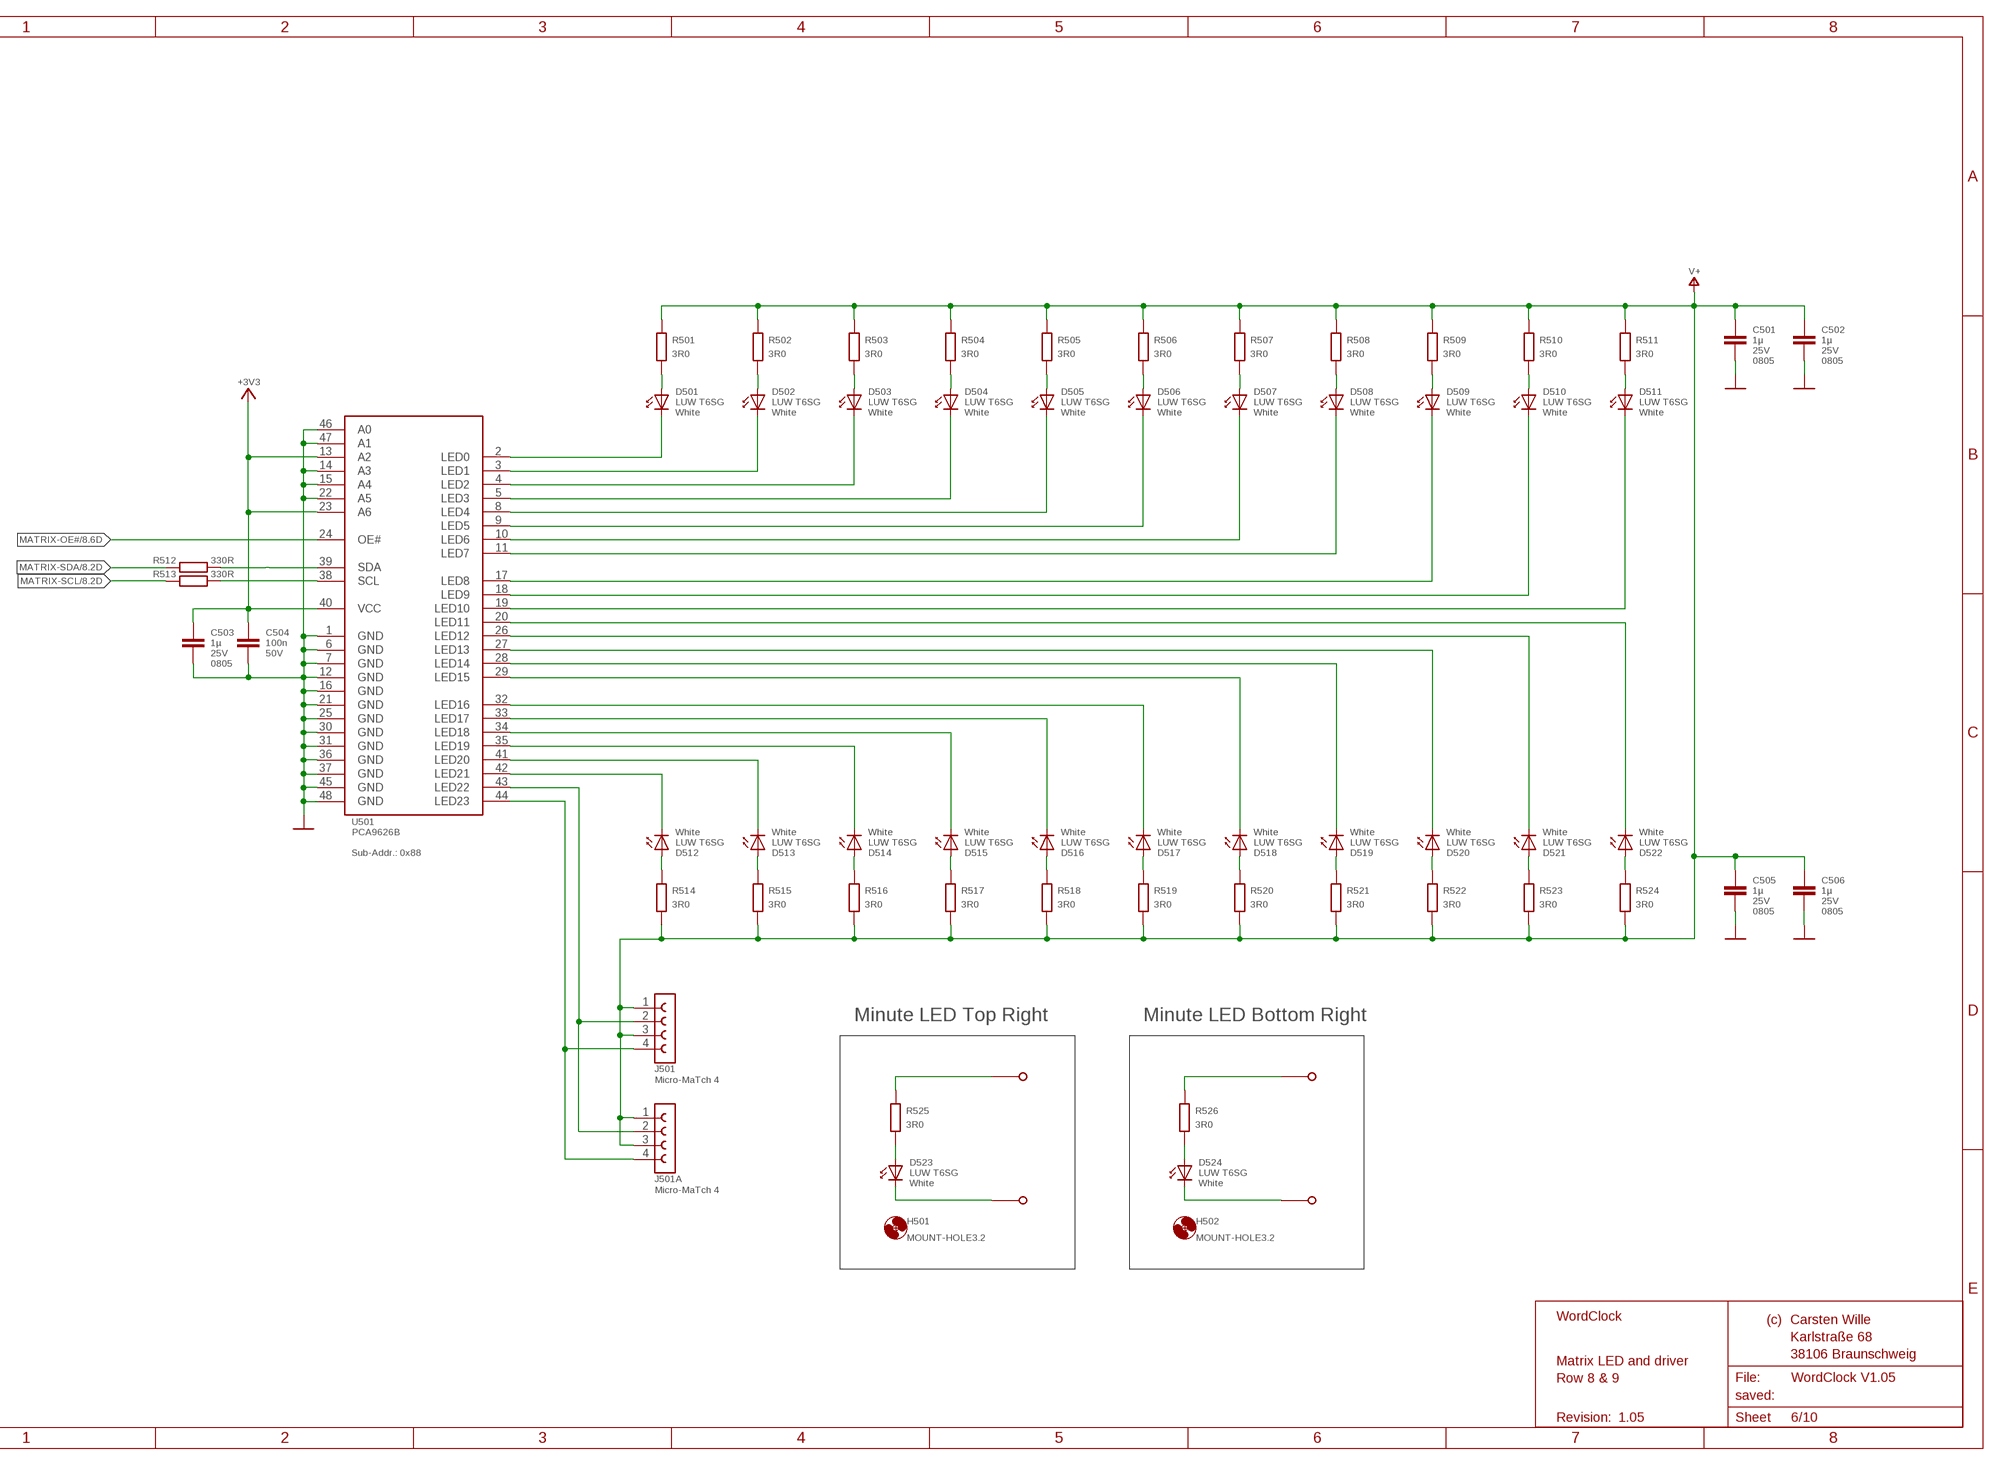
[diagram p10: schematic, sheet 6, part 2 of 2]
BLATT6 (BLATT-A3-LANDSCAPE_CW): SHEET_LINE1: Matrix LED and driver; SHEET_LINE2: Row 8 & 9

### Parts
C501  1E-6-1U-0805  [C0805]
C502  1E-6-1U-0805  [C0805]
C503  1E-6-1U-0805  [C0805]
C504  1E-9-100N-0603  [C0603]
C505  1E-6-1U-0805  [C0805]
C506  1E-6-1U-0805  [C0805]
D501  TOPLED-LUW  [P-LCC-2]
D502  TOPLED-LUW  [P-LCC-2]
D503  TOPLED-LUW  [P-LCC-2]
D504  TOPLED-LUW  [P-LCC-2]
D505  TOPLED-LUW  [P-LCC-2]
D506  TOPLED-LUW  [P-LCC-2]
D507  TOPLED-LUW  [P-LCC-2]
D508  TOPLED-LUW  [P-LCC-2]
D509  TOPLED-LUW  [P-LCC-2]
D510  TOPLED-LUW  [P-LCC-2]
D511  TOPLED-LUW  [P-LCC-2]
D512  TOPLED-LUW  [P-LCC-2]
D513  TOPLED-LUW  [P-LCC-2]
D514  TOPLED-LUW  [P-LCC-2]
D515  TOPLED-LUW  [P-LCC-2]
D516  TOPLED-LUW  [P-LCC-2]
D517  TOPLED-LUW  [P-LCC-2]
D518  TOPLED-LUW  [P-LCC-2]
D519  TOPLED-LUW  [P-LCC-2]
D520  TOPLED-LUW  [P-LCC-2]
D521  TOPLED-LUW  [P-LCC-2]
D522  TOPLED-LUW  [P-LCC-2]
D523  TOPLED-LUW  [P-LCC-2]
D524  TOPLED-LUW  [P-LCC-2]
H501  MOUNT-HOLE3.2  [3,2]
H502  MOUNT-HOLE3.2  [3,2]
J501  MICRO-MATCH-4  [MICRO-MATCH-4]
J501A  MICRO-MATCH-4  [MICRO-MATCH-4]
R501  1E0-3,0R-0603  [R0603]
R502  1E0-3,0R-0603  [R0603]
R503  1E0-3,0R-0603  [R0603]
R504  1E0-3,0R-0603  [R0603]
R505  1E0-3,0R-0603  [R0603]
R506  1E0-3,0R-0603  [R0603]
R507  1E0-3,0R-0603  [R0603]
R508  1E0-3,0R-0603  [R0603]
R509  1E0-3,0R-0603  [R0603]
R510  1E0-3,0R-0603  [R0603]
R511  1E0-3,0R-0603  [R0603]
R512  1E2-330R-0603  [R0603]
R513  1E2-330R-0603  [R0603]
R514  1E0-3,0R-0603  [R0603]
R515  1E0-3,0R-0603  [R0603]
R516  1E0-3,0R-0603  [R0603]
R517  1E0-3,0R-0603  [R0603]
R518  1E0-3,0R-0603  [R0603]
R519  1E0-3,0R-0603  [R0603]
R520  1E0-3,0R-0603  [R0603]
R521  1E0-3,0R-0603  [R0603]
R522  1E0-3,0R-0603  [R0603]
R523  1E0-3,0R-0603  [R0603]
R524  1E0-3,0R-0603  [R0603]
R525  1E0-3,0R-0603  [R0603]
R526  1E0-3,0R-0603  [R0603]
U501  PCA9626  [LQFP48]
X501  SINGLE-PIN-40MIL  [SINGLE-PIN_BIG]
X502  SINGLE-PIN-40MIL  [SINGLE-PIN_BIG]
X503  SINGLE-PIN-40MIL  [SINGLE-PIN_BIG]
X504  SINGLE-PIN-40MIL  [SINGLE-PIN_BIG]

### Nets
+3V3: C503.1 C504.1 U501.13(A2) U501.23(A6) U501.40(VCC) ; also sheet 2,3,4,5,7,8
GND: C501.2 C502.2 C503.2 C504.2 C505.2 C506.2 U501.1(GND) U501.6(GND) U501.7(GND) U501.12(GND) U501.14(A3) U501.15(A4) U501.16(GND) U501.21(GND) U501.22(A5) U501.25(GND) U501.30(GND) U501.31(GND) U501.36(GND) U501.37(GND) U501.45(GND) U501.46(A0) U501.47(A1) U501.48(GND) ; also sheet 2,3,4,5,7,8
LED0@U5: D501.C U501.2(LED0)
LED1@U5: D502.C U501.3(LED1)
LED2@U5: D503.C U501.4(LED2)
LED3@U5: D504.C U501.5(LED3)
LED4@U5: D505.C U501.8(LED4)
LED5@U5: D506.C U501.9(LED5)
LED6@U5: D507.C U501.10(LED6)
LED7@U5: D508.C U501.11(LED7)
LED8@U5: D509.C U501.17(LED8)
LED9@U5: D510.C U501.18(LED9)
LED10@U5: D511.C U501.19(LED10)
LED11@U5: D522.C U501.20(LED11)
LED12@U5: D521.C U501.26(LED12)
LED13@U5: D520.C U501.27(LED13)
LED14@U5: D519.C U501.28(LED14)
LED15@U5: D518.C U501.29(LED15)
LED16@U5: D517.C U501.32(LED16)
LED17@U5: D516.C U501.33(LED17)
LED18@U5: D515.C U501.34(LED18)
LED19@U5: D514.C U501.35(LED19)
LED20@U5: D513.C U501.41(LED20)
LED21@U5: D512.C U501.42(LED21)
MATRIX-OE#: U501.24(OE#) ; also sheet 2,3,4,5,8
MATRIX-SCL: R513.1 ; also sheet 2,3,4,5,8
MATRIX-SDA: R512.1 ; also sheet 2,3,4,5,8
N$19: D523.C X503.1
N$38: J501.2 J501A.2 U501.43(LED22)
N$40: D523.A R525.2
N$41: J501.4 J501A.4 U501.44(LED23)
N$42: R525.1 X501.1
N$44: R526.1 X502.1
N$45: D524.C X504.1
N$46: D524.A R526.2
R1@U5: D501.A R501.2
R2@U5: D502.A R502.2
R3@U5: D503.A R503.2
R4@U5: D504.A R504.2
R5@U5: D505.A R505.2
R6@U5: D506.A R506.2
R7@U5: D507.A R507.2
R8@U5: D508.A R508.2
R9@U5: D509.A R509.2
R10@U5: D510.A R510.2
R11@U5: D511.A R511.2
R12@U5: D512.A R514.1
R13@U5: D513.A R515.1
R14@U5: D514.A R516.1
R15@U5: D515.A R517.1
R16@U5: D516.A R518.1
R17@U5: D517.A R519.1
R18@U5: D518.A R520.1
R19@U5: D519.A R521.1
R20@U5: D520.A R522.1
R21@U5: D521.A R523.1
R22@U5: D522.A R524.1
SCL@U5: R513.2 U501.38(SCL)
SDA@U5: R512.2 U501.39(SDA)
V+: C501.1 C502.1 C505.1 C506.1 J501.1 J501.3 J501A.1 J501A.3 R501.1 R502.1 R503.1 R504.1 R505.1 R506.1 R507.1 R508.1 R509.1 R510.1 R511.1 R514.2 R515.2 R516.2 R517.2 R518.2 R519.2 R520.2 R521.2 R522.2 R523.2 R524.2 ; also sheet 2,3,4,5,7

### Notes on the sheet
- Sub-Addr.: 0x88
- Minute LED Top Right | Minute LED Bottom Right

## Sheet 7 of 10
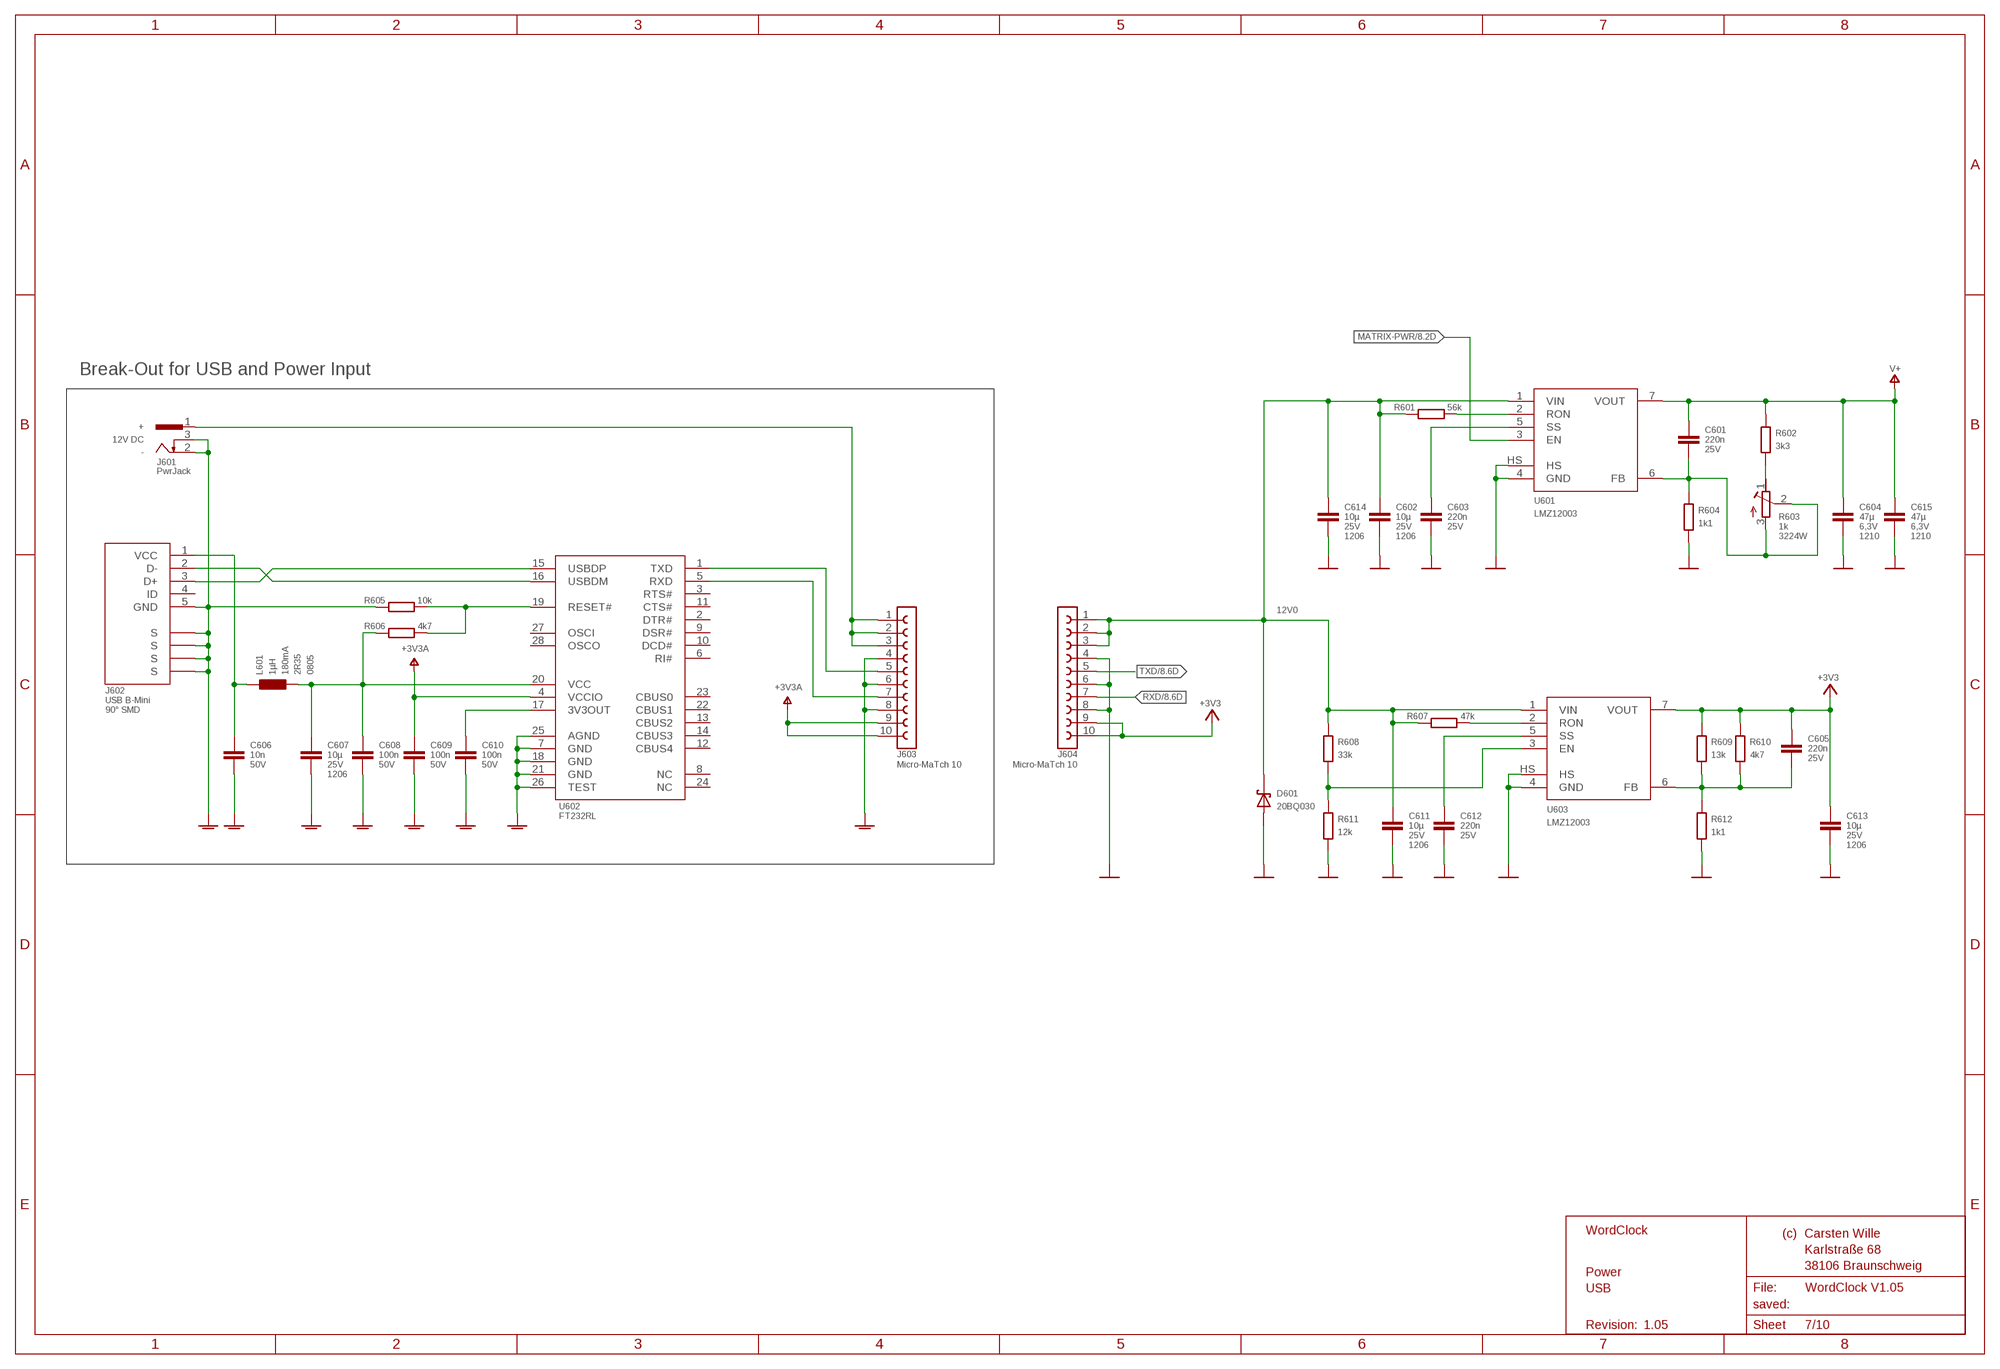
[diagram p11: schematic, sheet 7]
BLATT7 (BLATT-A3-LANDSCAPE_CW): SHEET_LINE1: Power; SHEET_LINE2: USB

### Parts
C601  1E-9-22N-0603  1E-9-220N-0603  [C0603]
C602  1E-6-10U-1206  [C1206]
C603  1E-9-22N-0603  1E-9-220N-0603  [C0603]
C604  1E-6-47U-1210  [C1210]
C605  1E-9-22N-0603  1E-9-220N-0603  [C0603]
C606  1E-9-10N-0603  [C0603]
C607  1E-6-10U-1206  [C1206]
C608  1E-9-100N-0603  [C0603]
C609  1E-9-100N-0603  [C0603]
C610  1E-9-100N-0603  [C0603]
C611  1E-6-10U-1206  [C1206]
C612  1E-9-22N-0603  1E-9-220N-0603  [C0603]
C613  1E-6-10U-1206  [C1206]
C614  1E-6-10U-1206  [C1206]
C615  1E-6-47U-1210  [C1210]
D601  20BQ030-SMB  [SMB]
J601  PWR-JACK  [RAPC722X]
J602  USB_B_MINI  [USB-MINI-B-SMD]
J603  MICRO-MATCH-10  [MICRO-MATCH-10]
J604  MICRO-MATCH-10  [MICRO-MATCH-10]
L601  L-1U0-0805  [L0805]
R601  1E4-56K-0603  [R0603]
R602  1E3-3,3K-0603  [R0603]
R603  R-TRIM1K-3224W  [RTRIM3224W]
R604  1E3-1,1K-0603  [R0603]
R605  1E4-10K-0603  [R0603]
R606  1E3-4,7K-0603  [R0603]
R607  1E4-47K-0603  [R0603]
R608  1E4-33K-0603  [R0603]
R609  1E4-13K-0603  [R0603]
R610  1E3-4,7K-0603  [R0603]
R611  1E4-12K-0603  [R0603]
R612  1E3-1,1K-0603  [R0603]
U601  LMZ12003  [TO-PMOD-7HS]
U602  FT232RL  [SSOP28]
U603  LMZ12003  [TO-PMOD-7HS]

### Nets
12V0: C602.1 C611.1 C614.1 D601.C J604.1 J604.2 J604.3 R601.1 R607.1 R608.1 U601.1(VIN) U603.1(VIN)
+3V3: C605.1 C613.1 J604.9 J604.10 R609.1 R610.1 U603.7(VOUT) ; also sheet 2,3,4,5,6,8
+3V3A: C609.1 J603.9 J603.10 U602.4(VCCIO)
D+: J602.3(D+) U602.15(USBDP)
D-: J602.2(D-) U602.16(USBDM)
GND: C602.2 C603.2 C604.2 C611.2 C612.2 C613.2 C614.2 C615.2 D601.A J604.4 J604.6 J604.8 R604.2 R611.2 R612.2 U601.4(GND) U601.HS U603.4(GND) U603.HS ; also sheet 2,3,4,5,6,8
GNDA: C606.2 C607.2 C608.2 C609.2 C610.2 J601.2 J601.3 J602.5(GND) J602.S0(S) J602.S1(S) J602.S2(S) J602.S3(S) J603.4 J603.6 J603.8 R605.1 U602.7(GND) U602.18(GND) U602.21(GND) U602.25(AGND) U602.26(TEST)
MATRIX-PWR: U601.3(EN) ; also sheet 8
N$3: R608.2 R611.1 U603.3(EN)
N$4: C605.2 R609.2 R610.2 R612.1 U603.6(FB)
N$5: C601.2 R603.2(S) R603.3(E) R604.1 U601.6(FB)
N$6: C603.1 U601.5(SS)
N$7: R601.2 U601.2(RON)
N$8: C612.1 U603.5(SS)
N$10: R607.2 U603.2(RON)
N$14: C610.1 U602.17(3V3OUT)
N$15: C607.1 C608.1 L601.2 R606.1 U602.20(VCC)
N$69: J601.1 J603.1 J603.2 J603.3
N$70: J603.5 U602.1(TXD)
N$71: J603.7 U602.5(RXD)
N$73: R602.2 R603.1(A)
N$87: C606.1 J602.1(VCC) L601.1
N$88: R605.2 R606.2 U602.19(RESET#)
RXD: J604.7 ; also sheet 8
TXD: J604.5 ; also sheet 8
V+: C601.1 C604.1 C615.1 R602.1 U601.7(VOUT) ; also sheet 2,3,4,5,6
Unconnected: J602.4(ID) U602.2(DTR#) U602.3(RTS#) U602.6(RI#) U602.8(NC) U602.9(DSR#) U602.10(DCD#) U602.11(CTS#) U602.12(CBUS4) U602.13(CBUS2) U602.14(CBUS3) U602.22(CBUS1) U602.23(CBUS0) U602.24(NC) U602.27(OSCI) U602.28(OSCO)

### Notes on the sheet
- Break-Out for USB and Power Input
- +
- 12V DC
- -

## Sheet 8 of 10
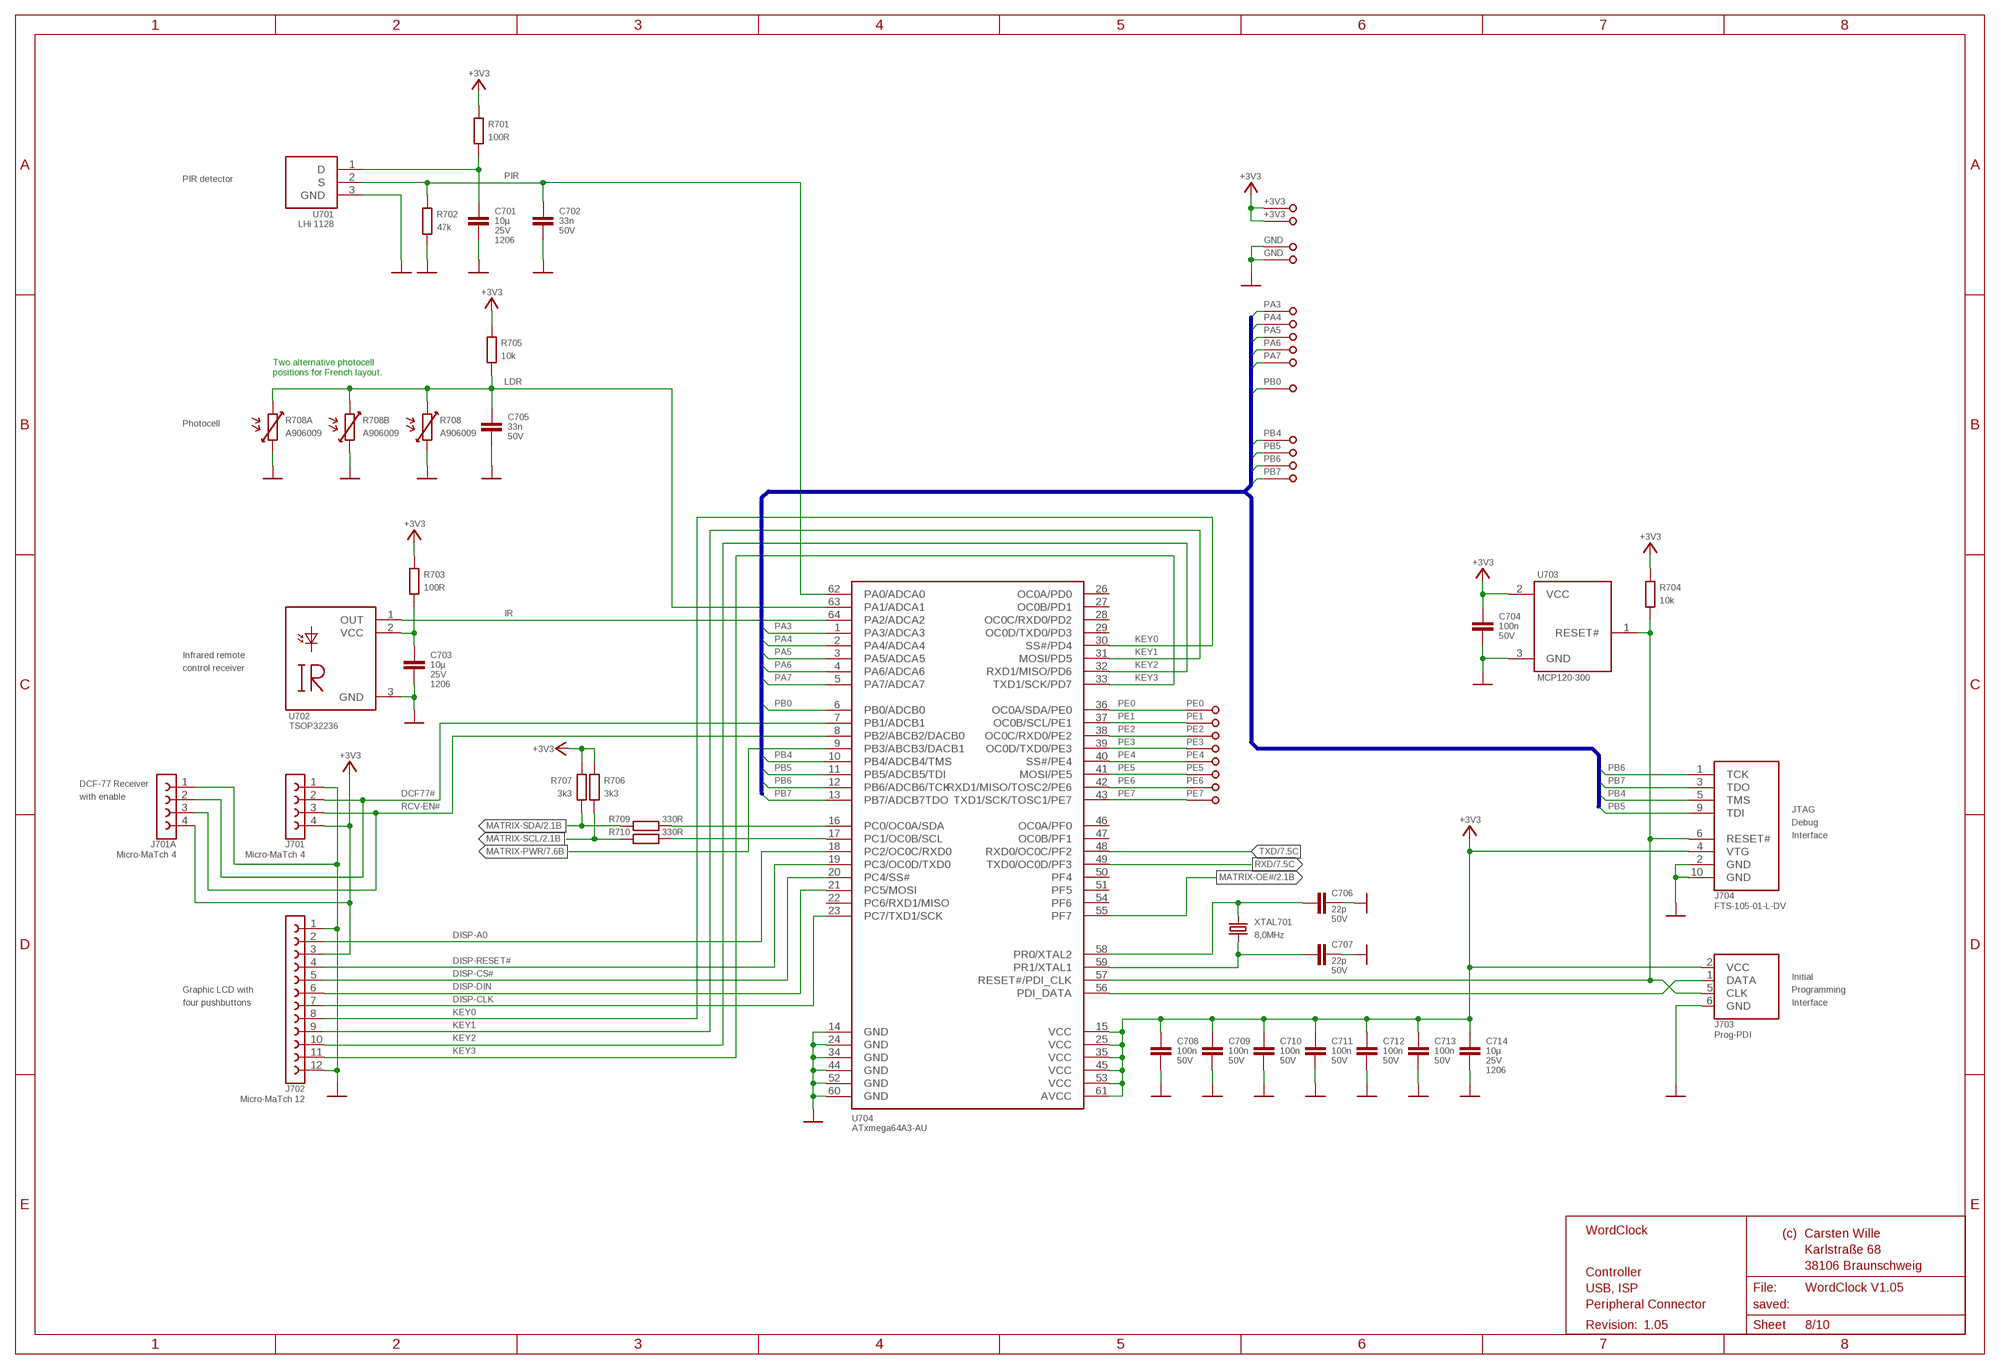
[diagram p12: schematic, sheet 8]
BLATT8 (BLATT-A3-LANDSCAPE_CW): SHEET_LINE1: Controller; SHEET_LINE2: USB, ISP; SHEET_LINE3: Peripheral Connector

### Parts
C701  1E-6-10U-1206  [C1206]
C702  1E-9-33N-0603  [C0603]
C703  1E-6-10U-1206  [C1206]
C704  1E-9-100N-0603  [C0603]
C705  1E-9-33N-0603  [C0603]
C706  1E-12-22P-0603  [C0603]
C707  1E-12-22P-0603  [C0603]
C708  1E-9-100N-0603  [C0603]
C709  1E-9-100N-0603  [C0603]
C710  1E-9-100N-0603  [C0603]
C711  1E-9-100N-0603  [C0603]
C712  1E-9-100N-0603  [C0603]
C713  1E-9-100N-0603  [C0603]
C714  1E-6-10U-1206  [C1206]
J701  MICRO-MATCH-4  [MICRO-MATCH-4]
J701A  MICRO-MATCH-4  [MICRO-MATCH-4]
J702  MICRO-MATCH-12  [MICRO-MATCH-12]
J703  PROG-PDI  [MA03-2]
J704  JTAG_ATMEL-50MIL  [FTS-105-01-L-DV]
R701  1E2-100R-0603  [R0603]
R702  1E4-47K-0603  [R0603]
R703  1E2-100R-0603  [R0603]
R704  1E4-10K-0603  [R0603]
R705  1E4-10K-0603  [R0603]
R706  1E3-3,3K-0603  [R0603]
R707  1E3-3,3K-0603  [R0603]
R708  LDR  [LDR_A90]
R708A  LDR  [LDR_A90]
R708B  LDR  [LDR_A90]
R709  1E2-330R-0603  [R0603]
R710  1E2-330R-0603  [R0603]
U701  LHI1128  [TO-5]
U702  TSOP32236  [TSOP322]
U703  MCP120  [SOT23]
U704  XMEGA64A3  [TQFP64]
X1  SINGLE-PIN-36MIL  [SINGLE-PIN]
X2  SINGLE-PIN-36MIL  [SINGLE-PIN]
X3  SINGLE-PIN-36MIL  [SINGLE-PIN]
X4  SINGLE-PIN-36MIL  [SINGLE-PIN]
X5  SINGLE-PIN-36MIL  [SINGLE-PIN]
X6  SINGLE-PIN-36MIL  [SINGLE-PIN]
X7  SINGLE-PIN-36MIL  [SINGLE-PIN]
X8  SINGLE-PIN-36MIL  [SINGLE-PIN]
X9  SINGLE-PIN-36MIL  [SINGLE-PIN]
X10  SINGLE-PIN-36MIL  [SINGLE-PIN]
X11  SINGLE-PIN-36MIL  [SINGLE-PIN]
X12  SINGLE-PIN-36MIL  [SINGLE-PIN]
X13  SINGLE-PIN-36MIL  [SINGLE-PIN]
X14  SINGLE-PIN-36MIL  [SINGLE-PIN]
X15  SINGLE-PIN-36MIL  [SINGLE-PIN]
X16  SINGLE-PIN-36MIL  [SINGLE-PIN]
X17  SINGLE-PIN-36MIL  [SINGLE-PIN]
X18  SINGLE-PIN-36MIL  [SINGLE-PIN]
X21  SINGLE-PIN-36MIL  [SINGLE-PIN]
X22  SINGLE-PIN-36MIL  [SINGLE-PIN]
X23  SINGLE-PIN-36MIL  [SINGLE-PIN]
X24  SINGLE-PIN-36MIL  [SINGLE-PIN]
XTAL701  MQ-8.000  [MQ]

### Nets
+3V3: C704.1 C708.1 C709.1 C710.1 C711.1 C712.1 C713.1 C714.1 J701.4 J701A.4 J702.3 J703.2(VCC) J704.4(VTG) R701.1 R703.1 R704.1 R705.1 R706.1 R707.1 U703.2(VCC) U704.15(VCC) U704.25(VCC) U704.35(VCC) U704.45(VCC) U704.53(VCC) U704.61(AVCC) X23.P$1 X24.P$1 ; also sheet 2,3,4,5,6,7
DCF77#: J701.2 J701A.2 U704.7(PB1/ADCB1)
DISP-A0: J702.2 U704.18(PC2/OC0C/RXD0)
DISP-CLK: J702.7 U704.23(PC7/TXD1/SCK)
DISP-CS#: J702.5 U704.20(PC4/SS#)
DISP-DIN: J702.6 U704.21(PC5/MOSI)
DISP-RESET#: J702.4 U704.19(PC3/OC0D/TXD0)
GND: C701.2 C702.2 C703.2 C704.2 C705.2 C706.2 C707.2 C708.2 C709.2 C710.2 C711.2 C712.2 C713.2 C714.2 J701.1 J701A.1 J702.1 J702.12 J703.6(GND) J704.2(GND) J704.10(GND) R702.2 R708.2 R708A.2 R708B.2 U701.3(GND) U702.3(GND) U703.3(GND) U704.14(GND) U704.24(GND) U704.34(GND) U704.44(GND) U704.52(GND) U704.60(GND) X21.P$1 X22.P$1 ; also sheet 2,3,4,5,6,7
IR: U702.1(OUT) U704.64(PA2/ADCA2)
KEY0: J702.8 U704.30(SS#/PD4)
KEY1: J702.9 U704.31(MOSI/PD5)
KEY2: J702.10 U704.32(RXD1/MISO/PD6)
KEY3: J702.11 U704.33(TXD1/SCK/PD7)
LDR: C705.1 R705.2 R708.1 R708A.1 R708B.1 U704.63(PA1/ADCA1)
MATRIX-OE#: U704.55(PF7) ; also sheet 2,3,4,5,6
MATRIX-PWR: U704.9(PB3/ABCB3/DACB1) ; also sheet 7
MATRIX-SCL: R706.2 R710.1 ; also sheet 2,3,4,5,6
MATRIX-SDA: R707.2 R709.1 ; also sheet 2,3,4,5,6
N$1: R709.2 U704.16(PC0/OC0A/SDA)
N$2: R710.2 U704.17(PC1/OC0B/SCL)
N$9: J703.1(DATA) U704.56(PDI_DATA)
N$11: J703.5(CLK) J704.6(RESET#) R704.2 U703.1(RESET#) U704.57(RESET#/PDI_CLK)
N$12: C707.1 U704.59(PR1/XTAL1) XTAL701.3
N$13: C706.1 U704.58(PR0/XTAL2) XTAL701.1
N$36: C701.1 R701.2 U701.1(D)
N$39: C703.1 R703.2 U702.2(VCC)
PA3: U704.1(PA3/ADCA3) X9.P$1
PA4: U704.2(PA4/ADCA4) X10.P$1
PA5: U704.3(PA5/ADCA5) X11.P$1
PA6: U704.4(PA6/ADCA6) X12.P$1
PA7: U704.5(PA7/ADCA7) X13.P$1
PB0: U704.6(PB0/ADCB0) X14.P$1
PB4: J704.5(TMS) U704.10(PB4/ADCB4/TMS) X15.P$1
PB5: J704.9(TDI) U704.11(PB5/ADCB5/TDI) X16.P$1
PB6: J704.1(TCK) U704.12(PB6/ADCB6/TCK) X17.P$1
PB7: J704.3(TDO) U704.13(PB7/ADCB7TDO) X18.P$1
PE0: U704.36(OC0A/SDA/PE0) X1.P$1
PE1: U704.37(OC0B/SCL/PE1) X2.P$1
PE2: U704.38(OC0C/RXD0/PE2) X3.P$1
PE3: U704.39(OC0D/TXD0/PE3) X4.P$1
PE4: U704.40(SS#/PE4) X5.P$1
PE5: U704.41(MOSI/PE5) X6.P$1
PE6: U704.42(RXD1/MISO/TOSC2/PE6) X7.P$1
PE7: U704.43(TXD1/SCK/TOSC1/PE7) X8.P$1
PIR: C702.1 R702.1 U701.2(S) U704.62(PA0/ADCA0)
RCV-EN#: J701.3 J701A.3 U704.8(PB2/ABCB2/DACB0)
RXD: U704.49(TXD0/OC0D/PF3) ; also sheet 7
TXD: U704.48(RXD0/OC0C/PF2) ; also sheet 7
Unconnected: U704.22(PC6/RXD1/MISO) U704.26(OC0A/PD0) U704.27(OC0B/PD1) U704.28(OC0C/RXD0/PD2) U704.29(OC0D/TXD0/PD3) U704.46(OC0A/PF0) U704.47(OC0B/PF1) U704.50(PF4) U704.51(PF5) U704.54(PF6)

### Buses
PA[3..7],PB[0..7],PC[0..1]

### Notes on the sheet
- PIR detector
- Two alternative photocell
  positions for French layout.
- Photocell
- Infrared remote
- control receiver
- DCF-77 Receiver
- with enable
- JTAG
- Debug
- Interface
- Initial
- Graphic LCD with | Programming
- four pushbuttons | Interface

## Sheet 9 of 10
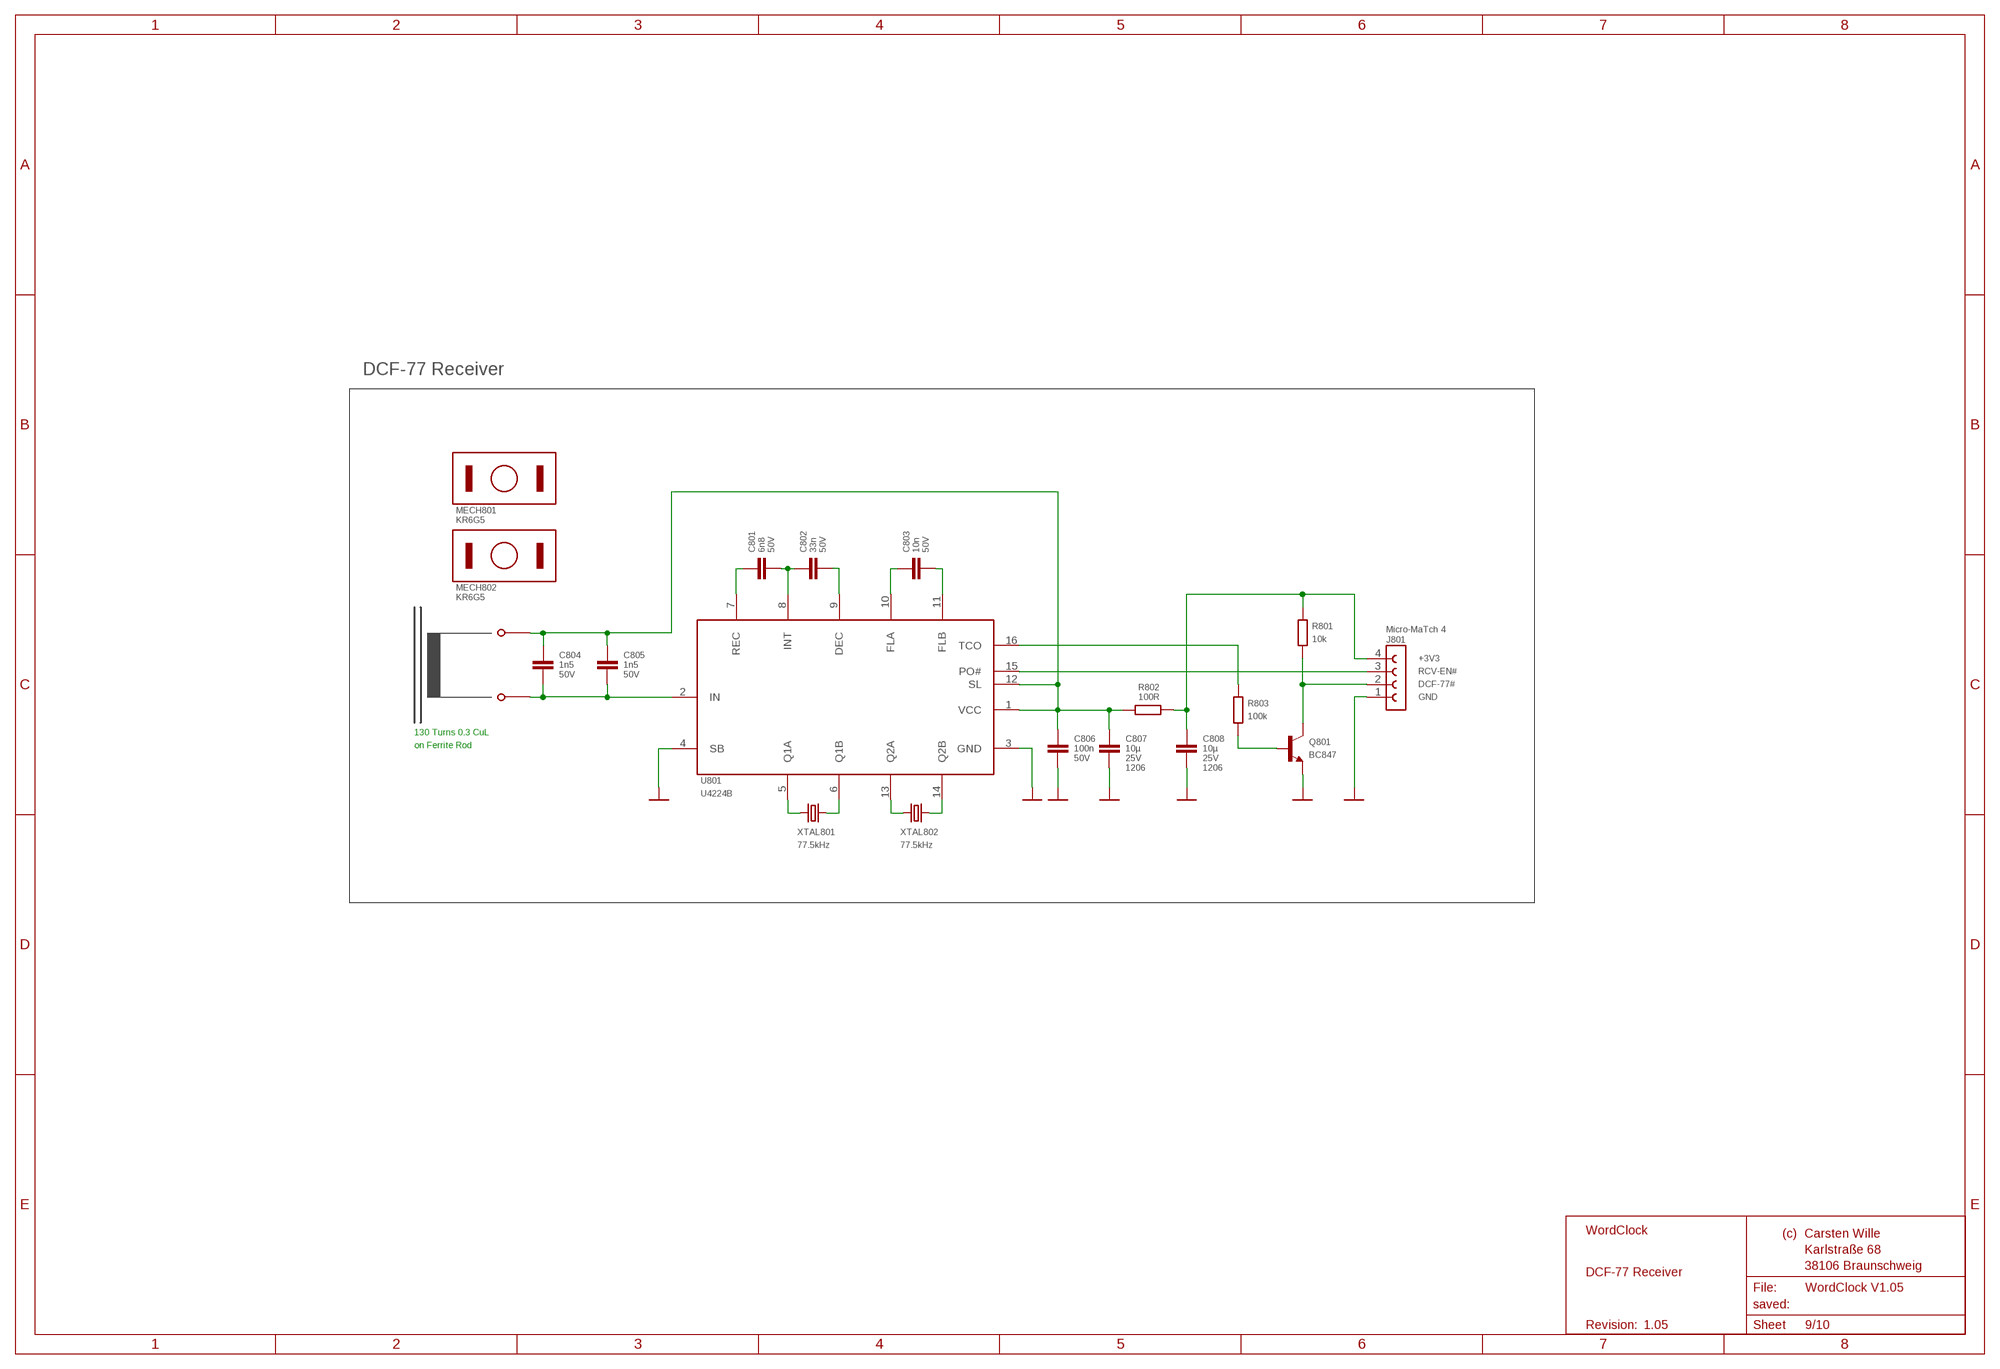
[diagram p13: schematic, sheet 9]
BLATT9 (BLATT-A3-LANDSCAPE_CW): SHEET_LINE1: DCF-77 Receiver

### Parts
C801  1E-9-6.8N-0603  [C0603]
C802  1E-9-33N-0603  [C0603]
C803  1E-9-10N-0603  [C0603]
C804  1E-9-1.5N-0603  [C0603]
C805  1E-9-1.5N-0603  [C0603]
C806  1E-9-100N-0603  [C0603]
C807  1E-6-10U-1206  [C1206]
C808  1E-6-10U-1206  [C1206]
J801  MICRO-MATCH-4  [MICRO-MATCH-4]
MECH801  SOCKET  [SOCKET]
MECH802  SOCKET  [SOCKET]
Q801  BC847  [SOT23]
R801  1E4-10K-0603  [R0603]
R802  1E2-100R-0603  [R0603]
R803  1E5-100K-0603  [R0603]
U801  U4224B  [SO16L]
X801  SINGLE-PIN-40MIL  [SINGLE-PIN_BIG]
X802  SINGLE-PIN-40MIL  [SINGLE-PIN_BIG]
XTAL801  TC26-77.5  [TC26H]
XTAL802  TC26-77.5  [TC26H]

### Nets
GND1: C806.2 C807.2 C808.2 J801.1 Q801.2(E) U801.3(GND) U801.4(SB) ; supply symbol labelled GND
N$16: U801.5(Q1A) XTAL801.2
N$20: U801.6(Q1B) XTAL801.1
N$21: U801.13(Q2A) XTAL802.2
N$22: U801.14(Q2B) XTAL802.1
N$23: C804.1 C805.1 C806.1 C807.1 R802.1 U801.1(VCC) U801.12(SL) X801.1
N$24: C808.1 J801.4 R801.1 R802.2
N$25: C801.1 U801.7(REC)
N$26: C801.2 C802.1 U801.8(INT)
N$27: C802.2 U801.9(DEC)
N$28: C803.1 U801.10(FLA)
N$29: C803.2 U801.11(FLB)
N$30: J801.3 U801.15(PO#)
N$31: C804.2 C805.2 U801.2(IN) X802.1
N$32: J801.2 Q801.3(C) R801.2
N$33: Q801.1(B) R803.2
N$34: R803.1 U801.16(TCO)

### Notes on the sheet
- DCF-77 Receiver
- +3V3
- RCV-EN#
- DCF-77#
- GND
- 130 Turns 0.3 CuL
- on Ferrite Rod

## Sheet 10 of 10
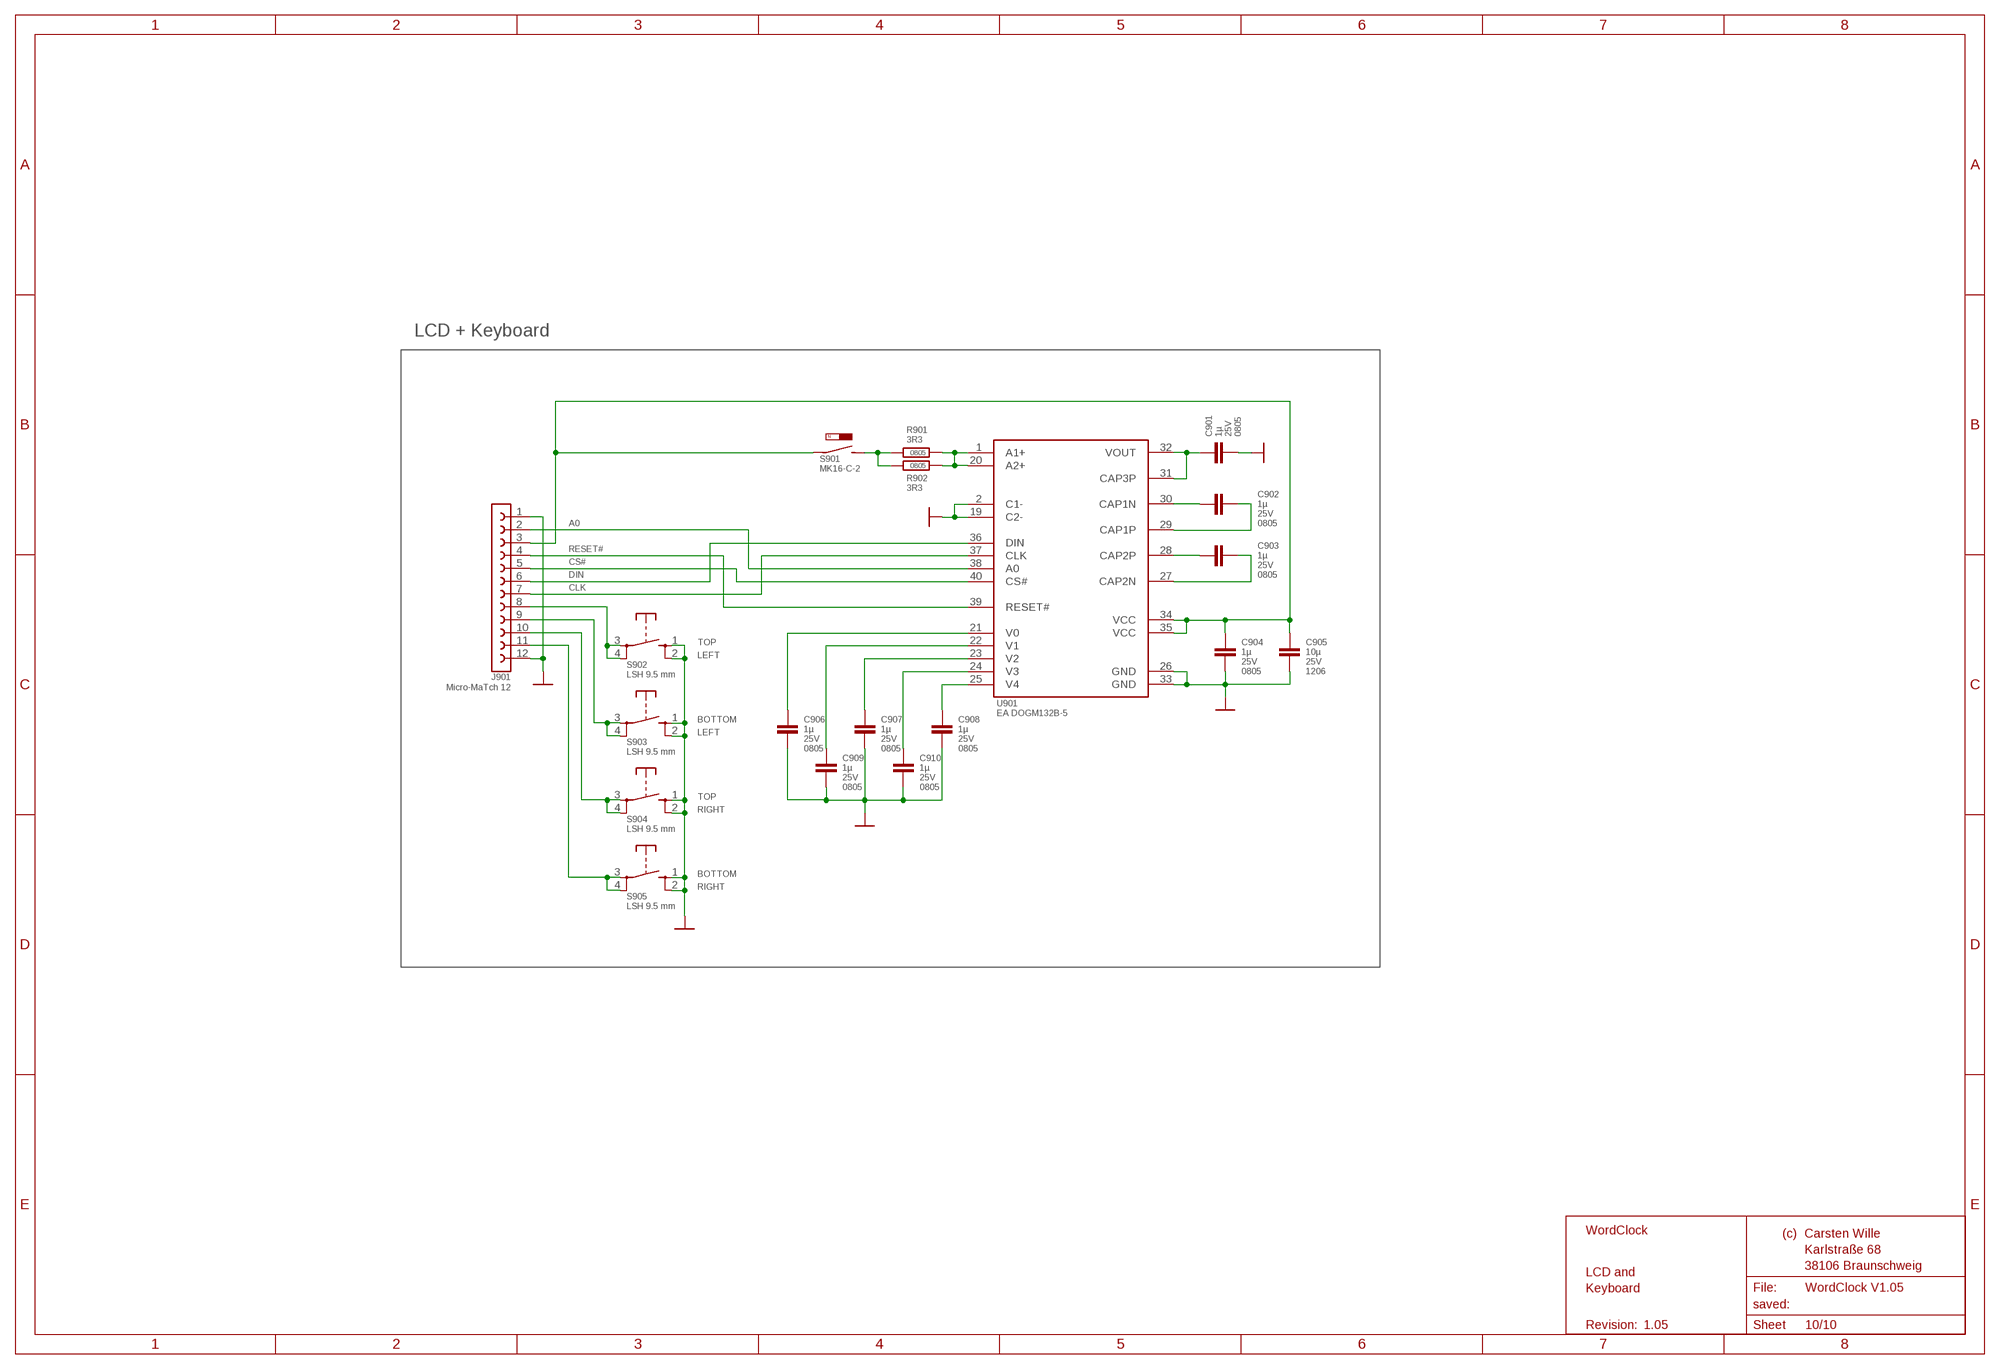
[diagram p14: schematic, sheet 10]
BLATT10 (BLATT-A3-LANDSCAPE_CW): SHEET_LINE1: LCD and; SHEET_LINE2: Keyboard

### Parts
C901  1E-6-1U-0805  [C0805]
C902  1E-6-1U-0805  [C0805]
C903  1E-6-1U-0805  [C0805]
C904  1E-6-1U-0805  [C0805]
C905  1E-6-10U-1206  [C1206]
C906  1E-6-1U-0805  [C0805]
C907  1E-6-1U-0805  [C0805]
C908  1E-6-1U-0805  [C0805]
C909  1E-6-1U-0805  [C0805]
C910  1E-6-1U-0805  [C0805]
J901  MICRO-MATCH-12  [MICRO-MATCH-12]
R901  1E0-3,3R-0805  [R0805]
R902  1E0-3,3R-0805  [R0805]
S901  MK16-SERIES  [MK16-X-2]
S902  LSH1301-9,5  [LSH1301]
S903  LSH1301-9,5  [LSH1301]
S904  LSH1301-9,5  [LSH1301]
S905  LSH1301-9,5  [LSH1301]
U901  EA_DOGM132B-5  [EA_DOGM132-5]

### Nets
A0: J901.2 U901.38(A0)
A+: R901.2 R902.2 U901.1(A1+) U901.20(A2+)
BL: J901.9 S903.3 S903.4
BR: J901.11 S905.3 S905.4
CLK: J901.7 U901.37(CLK)
CS#: J901.5 U901.40(CS#)
DIN: J901.6 U901.36(DIN)
GND2: C901.2 C904.2 C905.2 C906.2 C907.2 C908.2 C909.2 C910.2 J901.1 J901.12 S902.1 S902.2 S903.1 S903.2 S904.1 S904.2 S905.1 S905.2 U901.2(C1-) U901.19(C2-) U901.26(GND) U901.33(GND) ; supply symbol labelled GND
N$49: C903.2 U901.27(CAP2N)
N$50: C903.1 U901.28(CAP2P)
N$51: C902.2 U901.29(CAP1P)
N$52: C902.1 U901.30(CAP1N)
N$53: C901.1 U901.31(CAP3P) U901.32(VOUT)
RESET#: J901.4 U901.39(RESET#)
TL: J901.8 S902.3 S902.4
TR: J901.10 S904.3 S904.4
V0: C906.1 U901.21(V0)
V1: C909.1 U901.22(V1)
V2: C907.1 U901.23(V2)
V3: C910.1 U901.24(V3)
V4: C908.1 U901.25(V4)
VCC: C904.1 C905.1 J901.3 S901.2 U901.34(VCC) U901.35(VCC)
VCC+: R901.1 R902.1 S901.1

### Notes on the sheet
- LCD + Keyboard
- TOP
- LEFT
- BOTTOM
- LEFT
- TOP
- RIGHT
- BOTTOM
- RIGHT

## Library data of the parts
C101-C103 C105 C106 C201-C203 C205 C206 C301-C303 C305 C306 C401-C403 C405 C406 C501-C503 C505 C506 C901-C904 C906-C910 = o.Capacitor 0603 0805 1206:1E-6-*-?; MATERIAL: X7R; ORDER-MULTIPLE: 10; PACKAGE: 0805; SUPPLIER: Farnell; SUPPLIER-NUMBER: 145-8903; TOLERANCE: 10%; VAL: 1µ; VENDOR: Phycomp; VENDOR-NUMBER: 222291015663; VOLTAGE: 25V
C104 C204 C304 C404 C504 C608-C610 C704 C708-C713 C806 = o.Capacitor 0603 0805 1206:1E-9-*-?; MATERIAL: X7R; ORDER-MULTIPLE: 10; SUPPLIER: Farnell; SUPPLIER-NUMBER: 882-0023; TOLERANCE: 10%; VAL: 100n; VENDOR: Murata; VENDOR-NUMBER: GRM188R71H104KA93D; VOLTAGE: 50V
C601 C603 C605 C612 = o.Capacitor 0603 0805 1206:1E-9-*-?; MATERIAL: X7R; ORDER-MULTIPLE: 10; SUPPLIER: Farnell; SUPPLIER-NUMBER: 141-4626; TOLERANCE: 10%; VAL: 220n; VENDOR: Kemet; VENDOR-NUMBER: C0603C224K3RAC; VOLTAGE: 25V
C602 C607 C611 C613 C614 C701 C703 C714 C807 C808 C905 = o.Capacitor 0603 0805 1206:1E-6-*-?; MATERIAL: X7R; ORDER-MULTIPLE: 1; PACKAGE: 1206; SUPPLIER: Reichelt; SUPPLIER-NUMBER: X5R-G1206 10/25; TOLERANCE: 10%; VAL: 10µ; VOLTAGE: 25V
C604 C615 = o.Capacitor 0603 0805 1206.v6:1E-6-*-?; MATERIAL: Y5V; ORDER-MULTIPLE: 10; PACKAGE: 1210; SUPPLIER: Farnell; SUPPLIER-NUMBER: 1759367; TOLERANCE: +80%/-20%; VAL: 47µ; VENDOR: Multicomp; VENDOR-NUMBER: MCCA000491; VOLTAGE: 6,3V
C606 C803 = o.Capacitor 0603 0805 1206:1E-9-*-?; MATERIAL: X7R; ORDER-MULTIPLE: 10; SUPPLIER: Farnell; SUPPLIER-NUMBER: 165-0832; TOLERANCE: 10%; VAL: 10n; VENDOR: Kemet; VENDOR-NUMBER: C0603C103K5RAC; VOLTAGE: 50V
C702 C705 C802 = o.Capacitor 0603 0805 1206:1E-9-*-?; MATERIAL: X7R; ORDER-MULTIPLE: 10; SUPPLIER: Farnell; SUPPLIER-NUMBER: 141-4636; TOLERANCE: 10%; VAL: 33n; VENDOR: Kemet; VENDOR-NUMBER: C0603C333K5RAC; VOLTAGE: 50V
C706 C707 = o.Capacitor 0603 0805 1206:1E-12-*-?; MATERIAL: NP0; ORDER-MULTIPLE: 10; SUPPLIER: Farnell; SUPPLIER-NUMBER: 141-4622; TOLERANCE: 5%; VAL: 22p; VENDOR: Kemet; VENDOR-NUMBER: C0603C220J5GAC; VOLTAGE: 50V
C801 = o.Capacitor 0603 0805 1206:1E-9-*-?; MATERIAL: X7R; ORDER-MULTIPLE: 10; SUPPLIER: Farnell; SUPPLIER-NUMBER: 152-0266; TOLERANCE: 10%; VAL: 6n8; VENDOR: Kemet; VENDOR-NUMBER: C0603S682K5RAC; VOLTAGE: 50V
C804 C805 = o.Capacitor 0603 0805 1206:1E-9-*-?; MATERIAL: X7R; ORDER-MULTIPLE: 1; SUPPLIER: Reichelt; SUPPLIER-NUMBER: X7R-G0603 1,5N; TOLERANCE: 10%; VAL: 1n5; VENDOR: YAGEO; VENDOR-NUMBER: 06032R152K9BB0D; VOLTAGE: 50V
D101-D122 D201-D222 D301-D322 D401-D424 D501-D524 = o.Optical.v5:TOPLED: TOPLED; COLOR: White; SUPPLIER: RS Components; SUPPLIER-NUMBER: 664-8226; VAL: LUW T6SG; VENDOR: Osram; VENDOR-NUMBER: LUW T6SG-AABA-4N7Q
D601 = o.Semiconductor.v5:20BQ030: Schottky Diode, 2A, 30V; CURRENT: 2A; ORDER-MULTIPLE: 1; SUPPLIER: Farnell; SUPPLIER-NUMBER: 8647836; VAL: 20BQ030; VENDOR: Vishay; VENDOR-NUMBER: 20BQ030PBF; VOLTAGE: 30V
H401 H402 H501 H502 = holes:MOUNT-HOLE: MOUNTING HOLE with drill center marker
J401 J401A J501 J501A J701 J701A J801 = o.Connectors.v5:MICRO-MATCH-4: Micro-MaTch Board Connector Tyco female straight on board connector 4 pins.; SUPPLIER: Reichelt; SUPPLIER-NUMBER: MM FL 4G; VAL: Micro-MaTch 4; VENDOR: Tyco; VENDOR-NUMBER: 0-215079-4
J601 = o.Connectors.v5:PWR-JACK: Power-Jack; ORDER-MULTIPLE: 1; SUPPLIER: Farnell; SUPPLIER-NUMBER: 1608727; VAL: PwrJack; VENDOR: Switchcraft; VENDOR-NUMBER: RAPC722X
J602 = o.Connectors.v5:USB_B_MINI; SUPPLIER: Reichelt; SUPPLIER-NUMBER: USB BWM SMD; TYPE: 90° SMD; VAL: USB B-Mini; VENDOR: Assmann; VENDOR-NUMBER: A-USBB-M5/SMD
J603 J604 = o.Connectors.v5:MICRO-MATCH-10: Micro-MaTch Board Connector Tyco female straight on board connector 10 pins.; SUPPLIER: Reichelt; SUPPLIER-NUMBER: MM FL 10G; VAL: Micro-MaTch 10; VENDOR: Tyco; VENDOR-NUMBER: 1-215079-0
J702 J901 = o.Connectors.v5:MICRO-MATCH-12: Micro-MaTch Board Connector Tyco female straight on board connector 12 pins.; SUPPLIER: Reichelt; SUPPLIER-NUMBER: MM FL 12G; VAL: Micro-MaTch 12; VENDOR: Tyco; VENDOR-NUMBER: 1-215079-2
J703 = o.Connectors.v5:PROG-PDI; SUPPLIER: Farnell; SUPPLIER-NUMBER: 3418492; VAL: Prog-PDI; VENDOR: Tyco; VENDOR-NUMBER: 826632-3
J704 = o.Connectors.v6:JTAG_ATMEL; ORDER-MULTIPLE: 1; SUPPLIER: Farnell; SUPPLIER-NUMBER: 1667729; VAL: FTS-105-01-L-DV; VENDOR: Samtec; VENDOR-NUMBER: FTS-105-01-L-DV
L601 = o.Inductor:L-*-?; CURRENT: 180mA; PACKAGE: 0805; RESISTANCE: 2R35; SUPPLIER: Reichelt; SUPPLIER-NUMBER: L-0805AS 1,0µ; TOLERANCE: 5%; VAL: 1µH; VENDOR: FASTRON
MECH801 MECH802 = o.Mechanics:SOCKET: Fixing for calbe ties; SUPPLIER: Conrad; SUPPLIER-NUMBER: 540387; VAL: KR6G5; VENDOR: Hellermann Tyton; VENDOR-NUMBER: 151-24619
PCB1 = o.PCB Outlines.v6:PCB: PCB-Umrisse
Q801 = o.Semiconductor.v5:BC847; SUPPLIER: Farnell; SUPPLIER-NUMBER: 1081230; VAL: BC847; VENDOR: NXP; VENDOR-NUMBER: BC847
R101-R111 R114-R124 R201-R211 R214-R224 R301-R311 R314-R324 R401-R411 R414-R426 R501-R511 R514-R526 = o.Resistor 0603 0805 1206:1E0-*-?: 1R.. 9,1R; ORDER-MULTIPLE: 50; SUPPLIER: DigiKey; SUPPLIER-NUMBER: 541-3.00HCT-ND; TOLERANCE: 1%; VAL: 3R0; VENDOR: Vishay; VENDOR-NUMBER: CRCW06033.00FNEA; WATTAGE: 0,063W
R112 R113 R212 R213 R312 R313 R412 R413 R512 R513 R709 R710 = o.Resistor 0603 0805 1206:1E2-*-?: 100R.. 910R; ORDER-MULTIPLE: 50; SUPPLIER: Farnell; SUPPLIER-NUMBER: 933-1018; TOLERANCE: 1%; VAL: 330R; VENDOR: multicomp; VENDOR-NUMBER: MC 0.063W 0603 1% 330R; WATTAGE: 0,063W
R601 = o.Resistor 0603 0805 1206:1E4-*-?: 10k.. 91k; ORDER-MULTIPLE: 50; SUPPLIER: Farnell; SUPPLIER-NUMBER: 933-1360; TOLERANCE: 1%; VAL: 56k; VENDOR: multicomp; VENDOR-NUMBER: MC 0.063W 0603 1% 56k; WATTAGE: 0,063W
R602 R706 R707 = o.Resistor 0603 0805 1206:1E3-*-?: 1,0k.. 9,1k; ORDER-MULTIPLE: 50; SUPPLIER: Farnell; SUPPLIER-NUMBER: 933-1026; TOLERANCE: 1%; VAL: 3k3; VENDOR: multicomp; VENDOR-NUMBER: MC 0.063W 0603 1% 3k3; WATTAGE: 0,063W
R603 = o.Discrete.v6:R-TRIM: Trimming Potentiometer Status: unchecked; SUPPLIER: Farnell; SUPPLIER-NUMBER: 514871; TYPE: 3224W; VAL: 1k; VENDOR: Bourns; VENDOR-NUMBER: 3224W-001-102E
R604 R612 = o.Resistor 0603 0805 1206:1E3-*-?: 1,0k.. 9,1k; ORDER-MULTIPLE: 50; SUPPLIER: Farnell; SUPPLIER-NUMBER: 933-0445; TOLERANCE: 1%; VAL: 1k1; VENDOR: multicomp; VENDOR-NUMBER: MC 0.063W 0603 1% 1k1; WATTAGE: 0,063W
R605 R704 R705 R801 = o.Resistor 0603 0805 1206:1E4-*-?: 10k.. 91k; ORDER-MULTIPLE: 50; SUPPLIER: Farnell; SUPPLIER-NUMBER: 933-0399; TOLERANCE: 1%; VAL: 10k; VENDOR: multicomp; VENDOR-NUMBER: MC 0.063W 0603 1% 10k; WATTAGE: 0,063W
R606 R610 = o.Resistor 0603 0805 1206:1E3-*-?: 1,0k.. 9,1k; ORDER-MULTIPLE: 50; SUPPLIER: Farnell; SUPPLIER-NUMBER: 933-1247; TOLERANCE: 1%; VAL: 4k7; VENDOR: multicomp; VENDOR-NUMBER: MC 0.063W 0603 1% 4k7; WATTAGE: 0,063W
R607 R702 = o.Resistor 0603 0805 1206:1E4-*-?: 10k.. 91k; ORDER-MULTIPLE: 50; SUPPLIER: Farnell; SUPPLIER-NUMBER: 933-1255; TOLERANCE: 1%; VAL: 47k; VENDOR: multicomp; VENDOR-NUMBER: MC 0.063W 0603 1% 47k; WATTAGE: 0,063W
R608 = o.Resistor 0603 0805 1206:1E4-*-?: 10k.. 91k; ORDER-MULTIPLE: 50; SUPPLIER: Farnell; SUPPLIER-NUMBER: 933-1034; TOLERANCE: 1%; VAL: 33k; VENDOR: multicomp; VENDOR-NUMBER: MC 0.063W 0603 1% 33k; WATTAGE: 0,063W
R609 = o.Resistor 0603 0805 1206:1E4-*-?: 10k.. 91k; ORDER-MULTIPLE: 50; SUPPLIER: Farnell; SUPPLIER-NUMBER: 933-0569; TOLERANCE: 1%; VAL: 13k; VENDOR: multicomp; VENDOR-NUMBER: MC 0.063W 0603 1% 13k; WATTAGE: 0,063W
R611 = o.Resistor 0603 0805 1206:1E4-*-?: 10k.. 91k; ORDER-MULTIPLE: 50; SUPPLIER: Farnell; SUPPLIER-NUMBER: 933-0518; TOLERANCE: 1%; VAL: 12k; VENDOR: multicomp; VENDOR-NUMBER: MC 0.063W 0603 1% 12k; WATTAGE: 0,063W
R701 R703 R802 = o.Resistor 0603 0805 1206:1E2-*-?: 100R.. 910R; ORDER-MULTIPLE: 50; SUPPLIER: Farnell; SUPPLIER-NUMBER: 933-0364; TOLERANCE: 1%; VAL: 100R; VENDOR: multicomp; VENDOR-NUMBER: MC 0.063W 0603 1% 100R; WATTAGE: 0,063W
R708 R708A R708B = o.Discrete.v6:LDR: Photocell A 9060; SUPPLIER: Reichelt; SUPPLIER-NUMBER: LDR 07; VAL: A906009; VENDOR: PerkinElmer; VENDOR-NUMBER: A 9060 09
R803 = o.Resistor 0603 0805 1206:1E5-*-?: 100k.. 910k; ORDER-MULTIPLE: 50; SUPPLIER: Farnell; SUPPLIER-NUMBER: 933-0402; TOLERANCE: 1%; VAL: 100k; VENDOR: multicomp; VENDOR-NUMBER: MC 0.063W 0603 1% 100k; WATTAGE: 0,063W
R901 R902 = o.Resistor 0603 0805 1206:1E0-*-?: 1R.. 9,1R; ORDER-MULTIPLE: 50; PACKAGE: 0805; SUPPLIER: Farnell; SUPPLIER-NUMBER: 933-3096; TOLERANCE: 1%; VAL: 3R3; VENDOR: multicomp; VENDOR-NUMBER: MC 0.1W 0805 3R3; WATTAGE: 0,1W
S901 = o.Switches:MK16-SERIES; SUPPLIER: Farnell; SUPPLIER-NUMBER: 1079488; VAL: MK16-C-2; VENDOR: MEDER electronic; VENDOR-NUMBER: MK16-C-2
S902-S905 = o.Switches:LSH1301; SUPPLIER: Reichelt; SUPPLIER-NUMBER: TASTER9319; VAL: LSH 9.5 mm; VENDOR: Schurter; VENDOR-NUMBER: 1301.9319
U101 U201 U301 U401 U501 = o.Semiconductor.v5:PCA9626: 24-bit 100mA 40V LED Driver Status: unchecked; SUPPLIER: DigiKey; SUPPLIER-NUMBER: 568-4774-1-ND; VAL: PCA9626B; VENDOR: NXP; VENDOR-NUMBER: PCA9626B
U601 U603 = o.Semiconductor.v5:LMZ1*03: 3A Simple Switcher Power Module; IOUT: 3A; ORDER-MULTIPLE: 1; SUPPLIER: DigiKey; SUPPLIER-NUMBER: LMZ12003TZ-ADJCT-ND; VAL: LMZ12003; VENDOR: National Semiconductor; VENDOR-NUMBER: LMZ12003 TZ-ADJ; VIN: 4,5 -20V; VOUT: 0,8 - 6V
U602 = o.Controller.v5:FT232RL; SUPPLIER: Reichelt; SUPPLIER-NUMBER: FT 232 RL; VAL: FT232RL; VENDOR: FTDI Chip; VENDOR-NUMBER: FT232RL
U701 = o.Semiconductor.v5:LHI1128: Pyroelectric Detector LHi 1128; SUPPLIER: Reichelt; SUPPLIER-NUMBER: LHI 1128; VAL: LHi 1128; VENDOR: PerkinElmer; VENDOR-NUMBER: LHi 1128
U702 = o.Semiconductor.v5:TSOP322*; SUPPLIER: Farnell; SUPPLIER-NUMBER: 4913103; VAL: TSOP32236; VENDOR: Vishay; VENDOR-NUMBER: TSOP32236
U703 = o.Semiconductor.v5:MCP120: Microcontroller Supervisory Circuit with Open Drain Output; SUPPLIER: Farnell; SUPPLIER-NUMBER: 1292233; VAL: MCP120-300; VENDOR: Microchip; VENDOR-NUMBER: MCP120-300I/TT
U704 = o.Controller.v5:XMEGA*A3: ATxmega*A3-AU Status: unchecked; EEPROM: 2k; FLASH: 64k + 4k; SRAM: 4k; SUPPLIER: Farnell; SUPPLIER-NUMBER: 1748559; VAL: ATxmega64A3-AU; VENDOR: Atmel; VENDOR-NUMBER: ATxmega64A3-AU
U801 = o.Semiconductor.v5:U4224B: Time-Code Receiver with Digitized Serial Output The U4224B is a bipolar integrated striaght-through receiver circuit in the frequency range of 40 to 80 kHz. The device is designed for radio-controlled clock applications.; SUPPLIER: www.electronicpool.de; SUPPLIER-NUMBER: U4224B; VAL: U4224B; VENDOR: Temic; VENDOR-NUMBER: U4224B
U901 = o.Optical.v5:EA_DOGM132*-5; SUPPLIER: Reichelt; SUPPLIER-NUMBER: EA DOGM132B-5; VAL: EA DOGM132B-5; VENDOR: Electronic Assembly; VENDOR-NUMBER: EA DOGM132B-5
X1-X18 X21-X24 X401-X404 X501-X504 X801 X802 = o.Connectors.v5:SINGLE-PIN: Single-Pin
XTAL701 = o.Crystal.v5:MQ-*; SUPPLIER: Reichelt; SUPPLIER-NUMBER: 8,000000-MQ; VAL: 8,0MHz; VENDOR: Euroquartz; VENDOR-NUMBER: 8.000MHz MQ/30/30/40/12pF/60R
XTAL801 XTAL802 = o.Crystal.v5:TC26-*; SUPPLIER: Conrad; SUPPLIER-NUMBER: 168432-62; VAL: 77.5kHz; VENDOR: n/a; VENDOR-NUMBER: n/a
